(* Logix 5000 AddOnInstructionDefinition export Banner_R90C_R95C_R130C_Param_v4; software revision 33.00 *)

TYPE Banner_Hub_Discrete_Host_Out_Mirror_v4 :
STRUCT
   Mirroring_Enable : SINT;   // 0=Disabled, 1=Enabled.
   Mirroring_Port : SINT;   // 0=Port1, 1=Port2, 2=Port3, 3=Port4, Next set only for R95C 4=Port5, 5=Port6, 6=Port7, 7=Port8.
   Mirroring_Channel : SINT;   // 0=Discrete1, 1=Discrete2.
   Mirroring_Inversion : SINT;   // 0=Not Inverted, 1=Inverted.
   Mirroring_Polarity : SINT;   // 0=NPN Output, 1=PNP Output.
   Mirroring_Output_Type : SINT;   // 0=Output Open Collector, 1=Output Push Pull.
END_STRUCT
END_TYPE

TYPE Banner_Hub_IO_Metrics_v4 :
STRUCT
   Port_Discrete1_Count : DINT;
   Port_Discrete1_Duration : DINT;
   Port_Discrete1_Events_Per_Minute : DINT;
   Port_Discrete1_Totalizer : DINT;
   Port_Discrete2_Count : DINT;
   Port_Discrete2_Duration : DINT;
   Port_Discrete2_Events_Per_Minute : DINT;
   Port_Discrete2_Totalizer : DINT;
END_STRUCT
END_TYPE

TYPE Banner_Hub_Port_Config_B22_v4 :   // Data elements that are unique to the B22 version of the IO-Link Hub.
STRUCT
   Mirroring_Enable : SINT;   // 0 = Disabled, 1 = Enabled.
   Mirroring_Port_Selection : SINT;   // 0 = Port1, 1 = Port2, 2 = Port3, 3 = Prot4, 4 = Prot5, 5 = Port6, 6 = Port7, 7 = Port8.
   Mirroring_Channel_Selection : INT;   // 0 = Discrete 1, 1 = Discrete 2.
   Mirroring_Inversion : SINT;   // 0 = Not Inverted, 1 = Inverted.
END_STRUCT
END_TYPE

TYPE Banner_Hub_Port_Config_v4 :
STRUCT
   Discrete1_IO : INT;   // 0=NPN, 1=PNP
   Discrete1_Delay_Mode : INT;   // 0=Disabled,1=On Off Delay, 2=On OneShot, 3=Off OneShot, 4=On Pulse Stretcher, 5=Off Pulse Stretcher, 6=Totalizer, 7=Retriggerable On OneShot, 8=Retriggerable Off OneShot.
   Discrete1_Delay_Timer1 : DINT;
   Discrete1_Delay_Timer2 : DINT;
   Discrete1_B22_Options : Banner_Hub_Port_Config_B22_v4;
   Discrete2_IO : INT;   // 0=NPN, 1=PNP
   Discrete2_Delay_Mode : INT;   // 0=Disabled,1=On Off Delay, 2=On OneShot, 3=Off OneShot, 4=On Pulse Stretcher, 5=Off Pulse Stretcher, 6=Totalizer, 7=Retriggerable On OneShot, 8=Retriggerable Off OneShot.
   Discrete2_Delay_Timer1 : DINT;
   Discrete2_Delay_Timer2 : DINT;
   Discrete2_B22_Options : Banner_Hub_Port_Config_B22_v4;
   Mirroring_Enable : SINT;   // 0=Disabled, 1=Enabled.
   Mirroring_Port : SINT;   // 0=Port1, 1=Port2, 2=Port3, 3=Port4. Next set only for R95C 4=Port5, 5=Port6, 6=Port7, 7=Port8.
   Mirroring_Channel : SINT;   // 0=Discrete1, 1=Discrete2.
   Mirroring_Inversion : SINT;   // 0=Not Inverted, 1=Inverted.
END_STRUCT
END_TYPE

TYPE Banner_Hub_RD_v4 :   // UDT that stores the Write Data for a LM.
STRUCT
   Master_Cycle_Time : INT;
   Min_Cycle_Time : INT;
   M_Sequence_Capability : INT;
   IO_Link_Version_ID : INT;
   Process_Data_Input_Length : INT;
   Process_Data_Output_Length : INT;
   Combined_Vendor_ID : DINT;   // IO-Link Vendor ID
   Vendor_ID1 : INT;
   Vendor_ID2 : INT;
   Combined_Device_ID : DINT;   // IO-Link Device ID
   Device_ID1 : INT;
   Device_ID2 : INT;
   Device_ID3 : INT;
   Serial_Number : STRING;
   All_Time_Run_Time : DINT;   // Run Counter in 1/4 hr increments
   IO_Metrics : Banner_Hub_IO_Metrics_v4[9];
END_STRUCT
END_TYPE

TYPE Banner_Hub_SMR_Port_v4 :
STRUCT
   Discrete1 : SINT;   // 0 = Normal setting, 1 = Reset metrics.
   Discrete2 : SINT;   // 0 = Normal setting, 1 = Reset metrics.
   Discrete1_Reset_Count : DINT;   // Value that Counter is set to when a Reset Metrics operation is activated.
   Discrete2_Reset_Count : DINT;   // Value that Counter is set to when a Reset Metrics operation is activated.
END_STRUCT
END_TYPE

TYPE Banner_Hub_v4 :   // All of the parameters for a R90C, R95C, or R130C Hub.
STRUCT
   Initial_Global_Read : BOOL;   // Determines if all of the IO-Link data has been read into the PLC yet
   Command : INT;   // Value placed in here will activate a read or write to a specifc IO-Link Index
   Read : Banner_Hub_RD_v4;   // Read Only Data
   Write : Banner_Hub_WD_v4;   // Write Data
   Archive : Banner_Hub_WD_v4;   // Archive of Write Data
   Reset : BOOL;   // Resets AOI. This will force a complete parameter read of the sensor.
END_STRUCT
END_TYPE

TYPE Banner_Hub_VSC_v4 :
STRUCT
   PDin1_Metric : INT;   // 0=Disabled, 1=Count, 2=Duration, 3=Events Per Minute.
   PDin1_Port : INT;   // 0=Port 1, 1=Port 2, 2=Port 3, 3=Port 4. Only for R95 models 5=Port 6, 6=Port 7, 7=Port 8.
   PDin1_Channel : INT;   // 0=Discrete 1, 1 =Discrete 2.
   PDin2_Metric : INT;   // 0=Disabled, 1=Count, 2=Duration, 3=Events Per Minute.
   PDin2_Port : INT;   // 0=Port 1, 1=Port 2, 2=Port 3, 3=Port 4. Only for R95 models 5=Port 6, 6=Port 7, 7=Port 8.
   PDin2_Channel : INT;   // 0=Discrete 1, 1 =Discrete 2.
   PDin3_Metric : INT;   // 0=Disabled, 1=Count, 2=Duration, 3=Events Per Minute.
   PDin3_Port : INT;   // 0=Port 1, 1=Port 2, 2=Port 3, 3=Port 4. Only for R95 models 5=Port 6, 6=Port 7, 7=Port 8.
   PDin3_Channel : INT;   // 0=Discrete 1, 1 =Discrete 2.
   PDin4_Metric : INT;   // 0=Disabled, 1=Count, 2=Duration, 3=Events Per Minute.
   PDin4_Port : INT;   // 0=Port 1, 1=Port 2, 2=Port 3, 3=Port 4. Only for R95 models 5=Port 6, 6=Port 7, 7=Port 8.
   PDin4_Channel : INT;   // 0=Discrete 1, 1 =Discrete 2.
END_STRUCT
END_TYPE

TYPE Banner_Hub_WD_v4 :   // UDT that stores the Write Data for a LM.
STRUCT
   System_Command : INT;   // See IODD file for list of commands that can be activated via the System Command interface
   Parameter_Access_Lock : SINT;   // Write access to all parameters is prohibited while value is 1. Only this parameter can be adjusted when value is 1.
   Data_Storage_Lock : SINT;   // Automatic data storage is disabled when this value is equal to 1. Read access is not affected.
   Local_Parameterization_Lock : SINT;   // Parameterization via local control elements on device is disabled.
   Local_User_Interface_Lock : SINT;   // Operation of local user interface is disabled.
   Resettable_Run_Time : DINT;   // Run Counter in 1/4 hr increments
   VSC : Banner_Hub_VSC_v4;   // Vendor Specific Configuration R90C-4B21 and R95C-8B21 models.
   Process_Data_Grouping : SINT;   // R95-8B22 only. 0 = Group by Port, 1 = Group by Channel.
   All_Time_Run_Time_Event_Time : DINT;   // Event Time in 1/4 hr increments
   Resettable_Run_Time_Event_Time : DINT;   // Event Time in 1/4 hour increments
   SMR : Banner_Hub_SMR_Port_v4[10];   // Selectable Metric Reset.
   Port_Config : Banner_Hub_Port_Config_v4[10];
   Discrete_Host_Out_Mirroring : Banner_Hub_Discrete_Host_Out_Mirror_v4;
END_STRUCT
END_TYPE

TYPE Banner_IOL_Port_v4 :   // UDT that has all of the data items necessary to communicate with a specific Port on a IO-Link Master
STRUCT
   Port_Controlled : INT;   // Each bit represents a port on an IO-Link Master. Set to 1 to tell AOI to control that port.
   Port_Activate : INT;   // Each bit represents a port on an IO-Link Master. When ON that port will process any commands in queue.
   Port_Read : INT;   // Each bit represents a port on an IO-Link Master. Used to determine when device AOI has requested a Read command.
   Port_Write : INT;   // Each bit represents a port on an IO-Link Master. Used to determine when device AOI has requested a Write command.
   Port_RW_Complete : INT;   // Each bit represents a port on an IO-Link Master. Tells device AOI that Read or Write request has been completed.
   Port_Device_Read : INT;
   Data_Transfer : SINT[190];   // Array to transfer data from IO-Master to device AOIs.
END_STRUCT
END_TYPE

ADD_ON_INSTRUCTION Banner_R90C_R95C_R130C_Param_v4   (* revision 4.4, vendor Banner Engineering *)
// AOI to read and write parameter data to an IO-Link R90C-4K, R95C-8B21, R95C-8B22, or R130C-8B22 IO-Link Hub.
// Revision note:
// Added R130C.
VAR_IN_OUT
   Hub : Banner_Hub_v4; {required}
   Port_Data : Banner_IOL_Port_v4; {required}
END_VAR
VAR_INPUT
   Port : INT; {required}
   Type : INT; {required}   // 4 = R90C-4B21, 8 = R95C-8B21, 22 = R95-8B22
END_VAR
VAR
   Control : DINT; {access None}
   Global_Read_Command_Value : INT; {access None}
   Global_Write_Command_Value : INT; {access None}
   Command_Being_Processed : BOOL; {access None}
   Update_Archive : BOOL; {access None}
   Index_Write_Inprocess : INT; {access None}
   Index_Write_Control : INT; {access None}
   Temp_Excess_Gain : DINT; {access None}
   Inprocess_Index : DINT; {access None}
   Index2 : SINT; {access None}
   Index1 : SINT; {access None}
   Index4 : SINT; {access None}
   Index3 : SINT; {access None}
   Index6 : SINT; {access None}
   Index5 : SINT; {access None}
   Index7 : SINT; {access None}
END_VAR

ROUTINE Logic   (* ladder *)
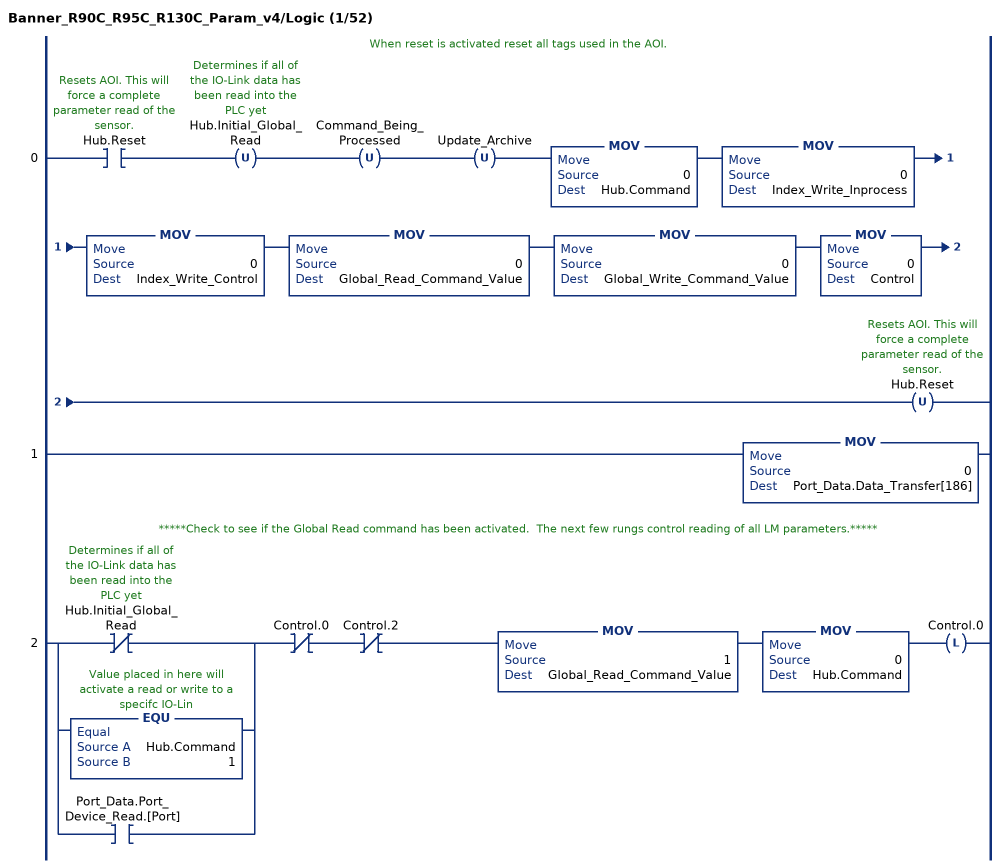
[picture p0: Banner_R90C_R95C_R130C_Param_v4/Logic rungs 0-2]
   // When reset is activated reset all tags used in the AOI.
   0: XIC(Hub.Reset)OTU(Hub.Initial_Global_Read)OTU(Command_Being_Processed)OTU(Update_Archive)MOV(0,Hub.Command)MOV(0,Index_Write_Inprocess)MOV(0,Index_Write_Control)MOV(0,Global_Read_Command_Value)MOV(0,Global_Write_Command_Value)MOV(0,Control)OTU(Hub.Reset);
   1: MOV(0,Port_Data.Data_Transfer[186]);
   // *****Check to see if the Global Read command has been activated.  The next few rungs control reading of all LM parameters.*****
   2: [XIO(Hub.Initial_Global_Read) ,EQU(Hub.Command,1) ,XIC(Port_Data.Port_Device_Read.[Port]) ]XIO(Control.0)XIO(Control.2)MOV(1,Global_Read_Command_Value)MOV(0,Hub.Command)OTL(Control.0);
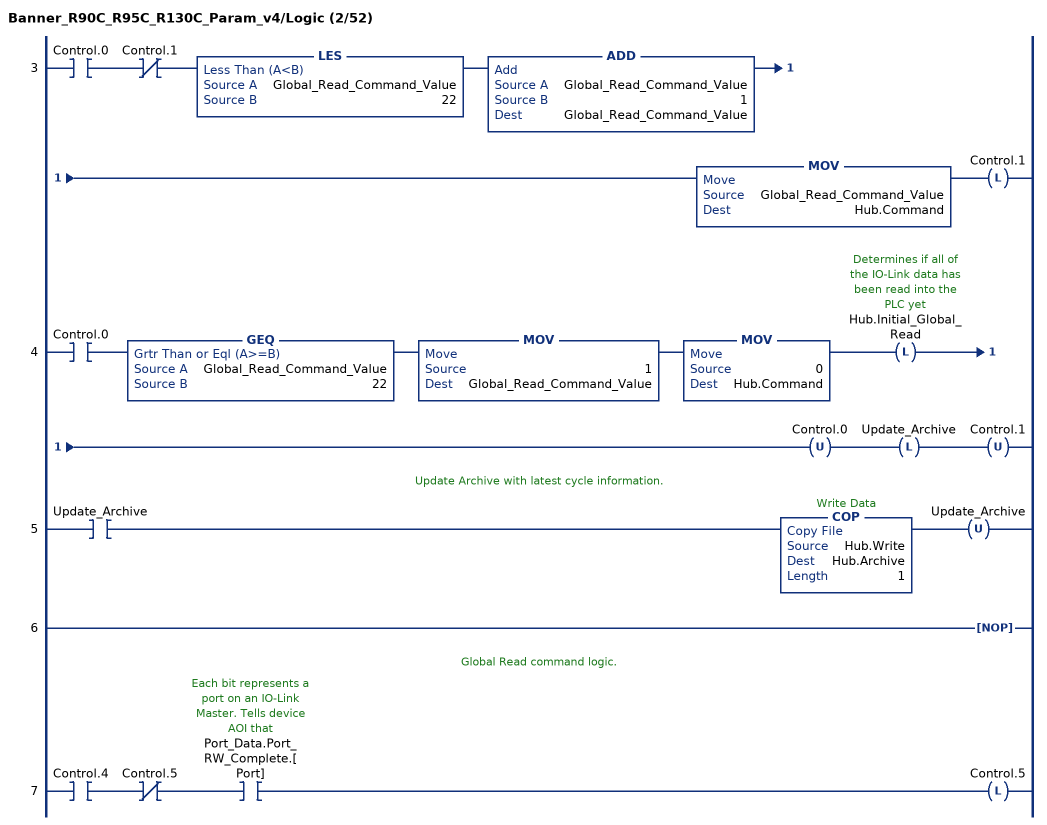
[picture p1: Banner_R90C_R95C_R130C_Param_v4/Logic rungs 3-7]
   3: XIC(Control.0)XIO(Control.1)LES(Global_Read_Command_Value,22)ADD(Global_Read_Command_Value,1,Global_Read_Command_Value)MOV(Global_Read_Command_Value,Hub.Command)OTL(Control.1);
   4: XIC(Control.0)GEQ(Global_Read_Command_Value,22)MOV(1,Global_Read_Command_Value)MOV(0,Hub.Command)OTL(Hub.Initial_Global_Read)OTU(Control.0)OTL(Update_Archive)OTU(Control.1);
   // Update Archive with latest cycle information.
   5: XIC(Update_Archive)COP(Hub.Write,Hub.Archive,1)OTU(Update_Archive);
   6: NOP();
   // Global Read command logic.
   7: XIC(Control.4)XIO(Control.5)XIC(Port_Data.Port_RW_Complete.[Port])OTL(Control.5);
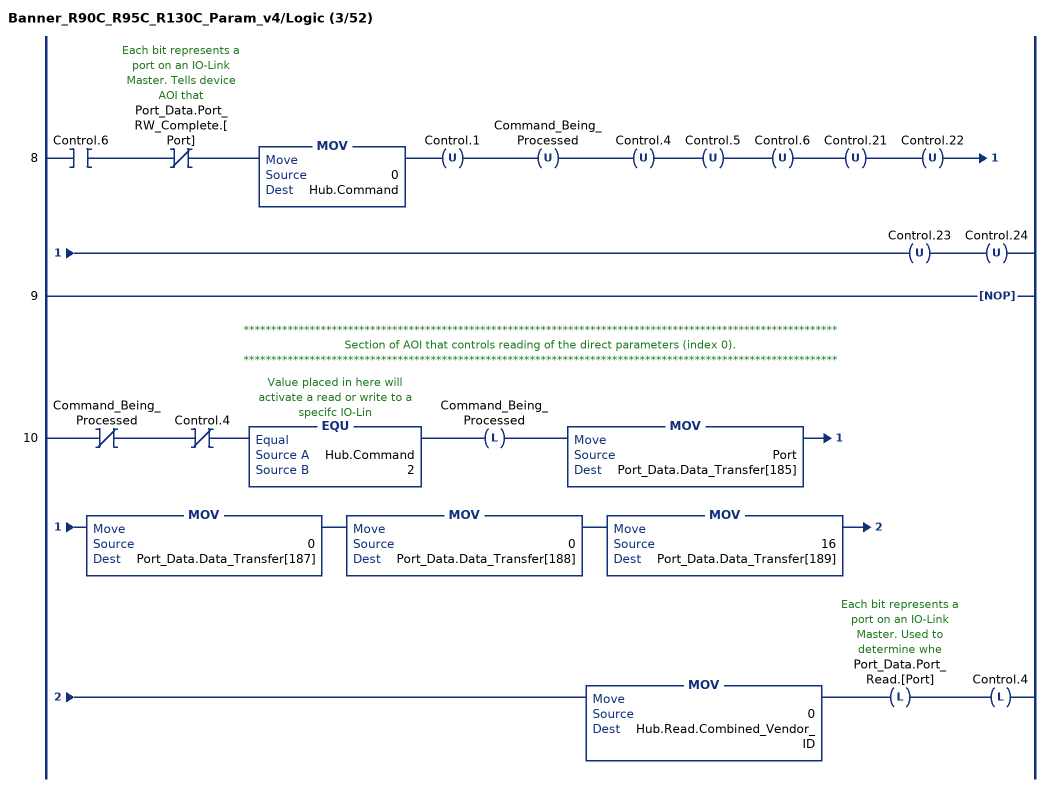
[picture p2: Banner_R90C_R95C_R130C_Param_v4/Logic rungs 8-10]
   8: XIC(Control.6)XIO(Port_Data.Port_RW_Complete.[Port])MOV(0,Hub.Command)OTU(Control.1)OTU(Command_Being_Processed)OTU(Control.4)OTU(Control.5)OTU(Control.6)OTU(Control.21)OTU(Control.22)OTU(Control.23)OTU(Control.24);
   9: NOP();
   // ************************************************************************************************************
   // Section of AOI that controls reading of the direct parameters (index 0).
   // ************************************************************************************************************
   10: XIO(Command_Being_Processed)XIO(Control.4)EQU(Hub.Command,2)OTL(Command_Being_Processed)MOV(Port,Port_Data.Data_Transfer[185])MOV(0,Port_Data.Data_Transfer[187])MOV(0,Port_Data.Data_Transfer[188])MOV(16,Port_Data.Data_Transfer[189])MOV(0,Hub.Read.Combined_Vendor_ID)OTL(Port_Data.Port_Read.[Port])OTL(Control.4);
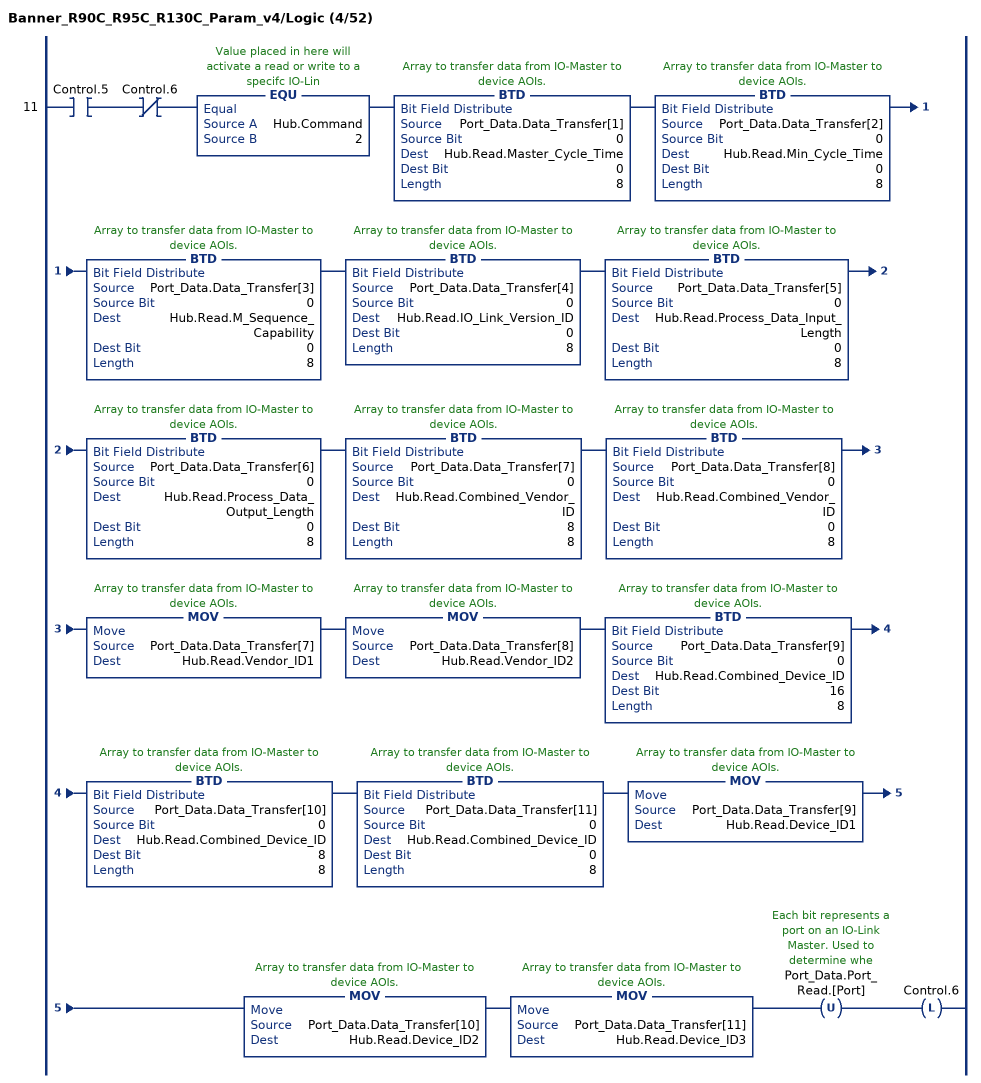
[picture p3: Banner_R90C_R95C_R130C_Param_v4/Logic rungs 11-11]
   11: XIC(Control.5)XIO(Control.6)EQU(Hub.Command,2)BTD(Port_Data.Data_Transfer[1],0,Hub.Read.Master_Cycle_Time,0,8)BTD(Port_Data.Data_Transfer[2],0,Hub.Read.Min_Cycle_Time,0,8)BTD(Port_Data.Data_Transfer[3],0,Hub.Read.M_Sequence_Capability,0,8)BTD(Port_Data.Data_Transfer[4],0,Hub.Read.IO_Link_Version_ID,0,8)BTD(Port_Data.Data_Transfer[5],0,Hub.Read.Process_Data_Input_Length,0,8)BTD(Port_Data.Data_Transfer[6],0,Hub.Read.Process_Data_Output_Length,0,8)BTD(Port_Data.Data_Transfer[7],0,Hub.Read.Combined_Vendor_ID,8,8)BTD(Port_Data.Data_Transfer[8],0,Hub.Read.Combined_Vendor_ID,0,8)MOV(Port_Data.Data_Transfer[7],Hub.Read.Vendor_ID1)MOV(Port_Data.Data_Transfer[8],Hub.Read.Vendor_ID2)BTD(Port_Data.Data_Transfer[9],0,Hub.Read.Combined_Device_ID,16,8)BTD(Port_Data.Data_Transfer[10],0,Hub.Read.Combined_Device_ID,8,8)BTD(Port_Data.Data_Transfer[11],0,Hub.Read.Combined_Device_ID,0,8)MOV(Port_Data.Data_Transfer[9],Hub.Read.Device_ID1)MOV(Port_Data.Data_Transfer[10],Hub.Read.Device_ID2)MOV(Port_Data.Data_Transfer[11],Hub.Read.Device_ID3)OTU(Port_Data.Port_Read.[Port])OTL(Control.6);
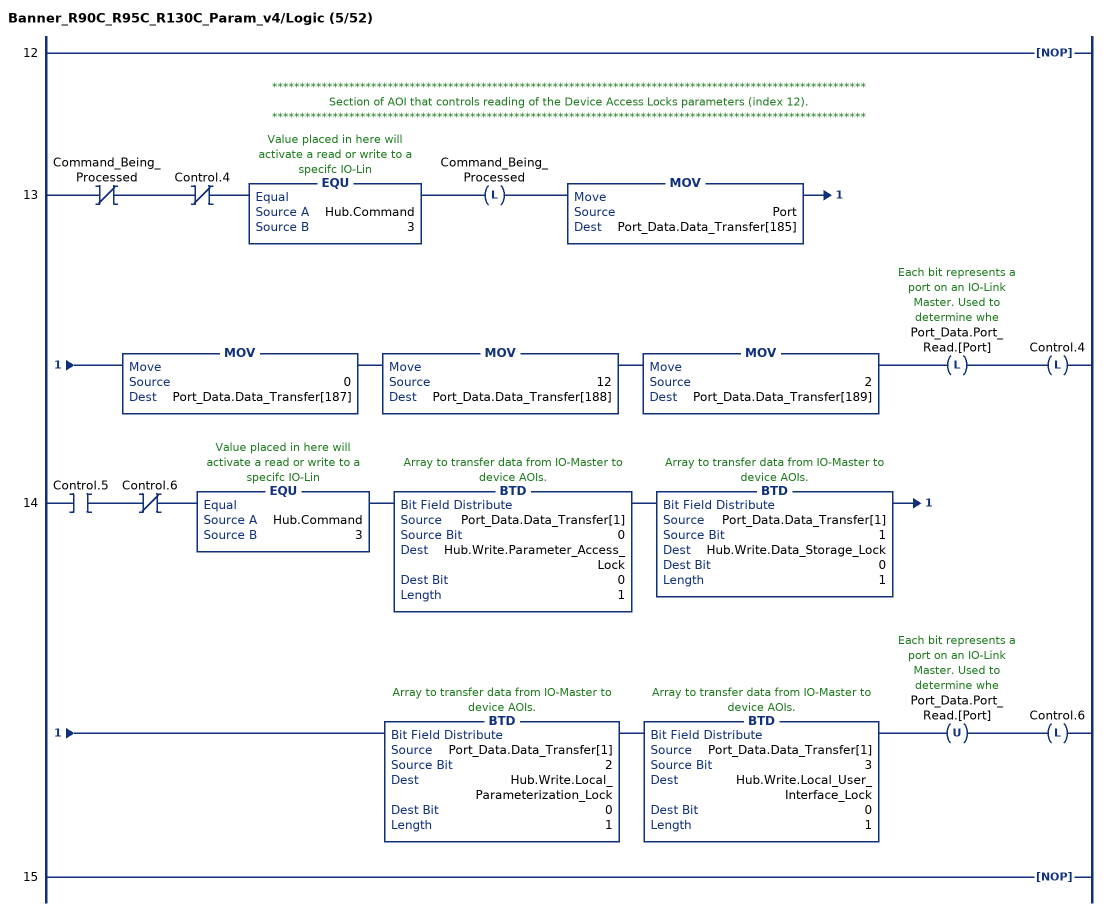
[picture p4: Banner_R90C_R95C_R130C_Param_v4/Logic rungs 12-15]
   12: NOP();
   // ************************************************************************************************************
   // Section of AOI that controls reading of the Device Access Locks parameters (index 12).
   // ************************************************************************************************************
   13: XIO(Command_Being_Processed)XIO(Control.4)EQU(Hub.Command,3)OTL(Command_Being_Processed)MOV(Port,Port_Data.Data_Transfer[185])MOV(0,Port_Data.Data_Transfer[187])MOV(12,Port_Data.Data_Transfer[188])MOV(2,Port_Data.Data_Transfer[189])OTL(Port_Data.Port_Read.[Port])OTL(Control.4);
   14: XIC(Control.5)XIO(Control.6)EQU(Hub.Command,3)BTD(Port_Data.Data_Transfer[1],0,Hub.Write.Parameter_Access_Lock,0,1)BTD(Port_Data.Data_Transfer[1],1,Hub.Write.Data_Storage_Lock,0,1)BTD(Port_Data.Data_Transfer[1],2,Hub.Write.Local_Parameterization_Lock,0,1)BTD(Port_Data.Data_Transfer[1],3,Hub.Write.Local_User_Interface_Lock,0,1)OTU(Port_Data.Port_Read.[Port])OTL(Control.6);
   15: NOP();
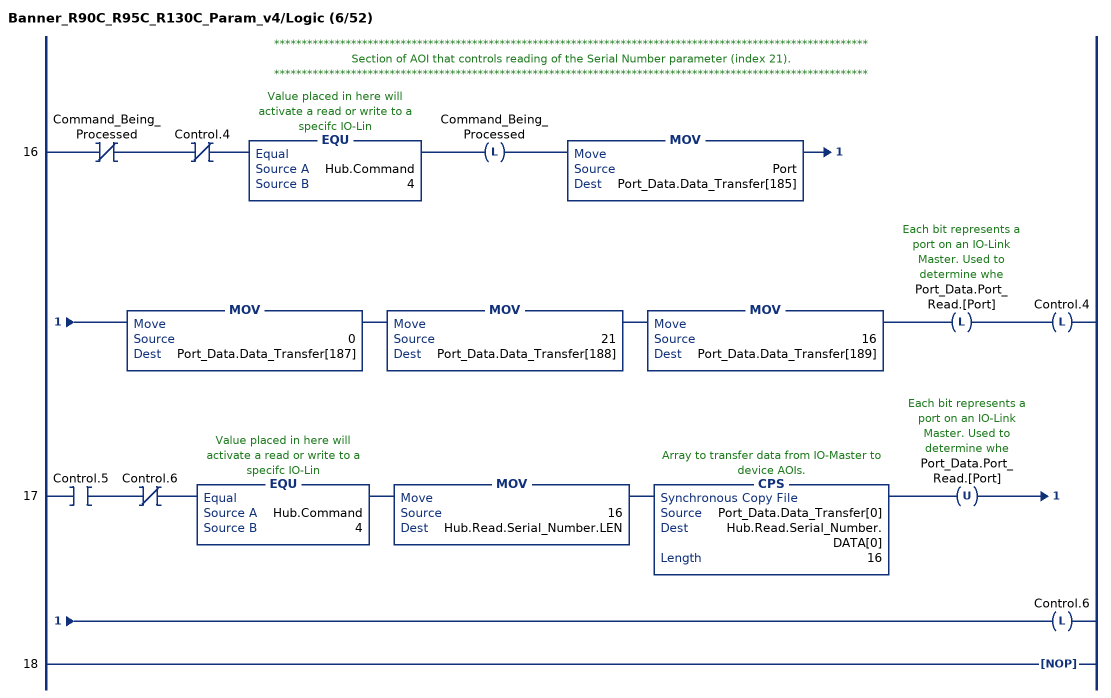
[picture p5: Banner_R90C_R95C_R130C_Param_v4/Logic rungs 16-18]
   // ************************************************************************************************************
   // Section of AOI that controls reading of the Serial Number parameter (index 21).
   // ************************************************************************************************************
   16: XIO(Command_Being_Processed)XIO(Control.4)EQU(Hub.Command,4)OTL(Command_Being_Processed)MOV(Port,Port_Data.Data_Transfer[185])MOV(0,Port_Data.Data_Transfer[187])MOV(21,Port_Data.Data_Transfer[188])MOV(16,Port_Data.Data_Transfer[189])OTL(Port_Data.Port_Read.[Port])OTL(Control.4);
   17: XIC(Control.5)XIO(Control.6)EQU(Hub.Command,4)MOV(16,Hub.Read.Serial_Number.LEN)CPS(Port_Data.Data_Transfer[0],Hub.Read.Serial_Number.DATA[0],16)OTU(Port_Data.Port_Read.[Port])OTL(Control.6);
   18: NOP();
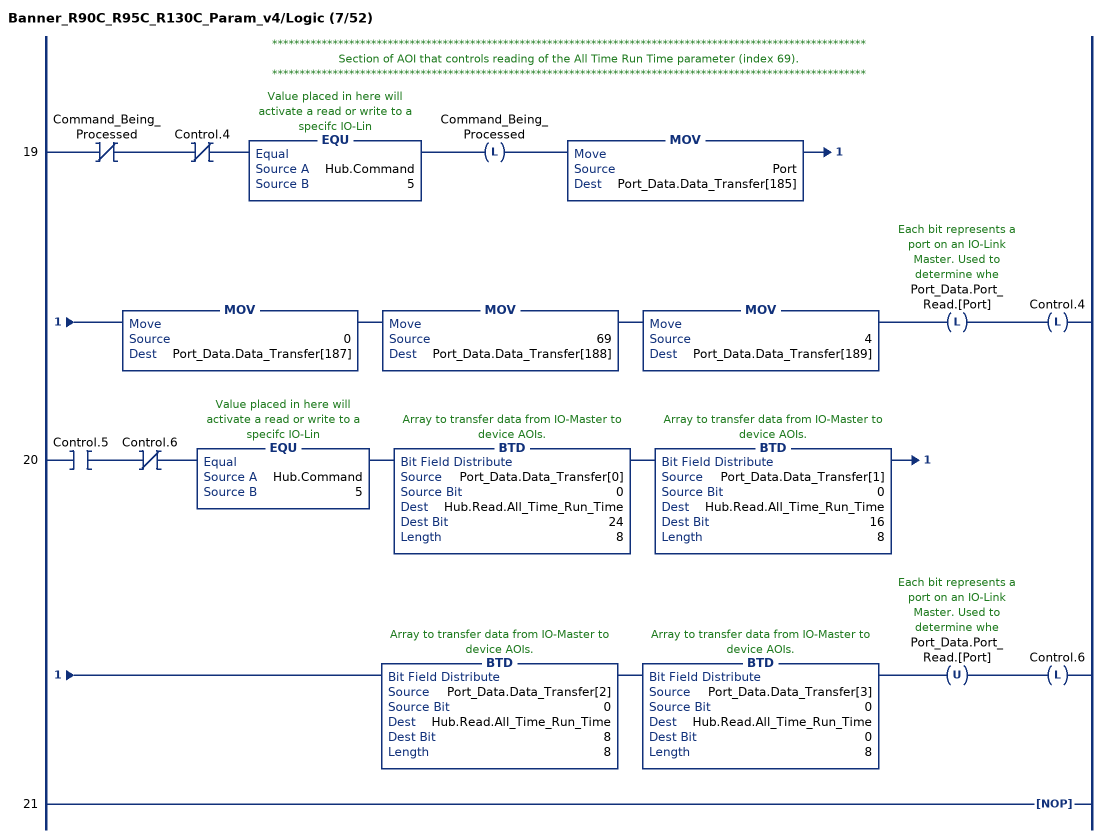
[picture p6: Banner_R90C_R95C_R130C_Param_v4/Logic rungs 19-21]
   // ************************************************************************************************************
   // Section of AOI that controls reading of the All Time Run Time parameter (index 69).
   // ************************************************************************************************************
   19: XIO(Command_Being_Processed)XIO(Control.4)EQU(Hub.Command,5)OTL(Command_Being_Processed)MOV(Port,Port_Data.Data_Transfer[185])MOV(0,Port_Data.Data_Transfer[187])MOV(69,Port_Data.Data_Transfer[188])MOV(4,Port_Data.Data_Transfer[189])OTL(Port_Data.Port_Read.[Port])OTL(Control.4);
   20: XIC(Control.5)XIO(Control.6)EQU(Hub.Command,5)BTD(Port_Data.Data_Transfer[0],0,Hub.Read.All_Time_Run_Time,24,8)BTD(Port_Data.Data_Transfer[1],0,Hub.Read.All_Time_Run_Time,16,8)BTD(Port_Data.Data_Transfer[2],0,Hub.Read.All_Time_Run_Time,8,8)BTD(Port_Data.Data_Transfer[3],0,Hub.Read.All_Time_Run_Time,0,8)OTU(Port_Data.Port_Read.[Port])OTL(Control.6);
   21: NOP();
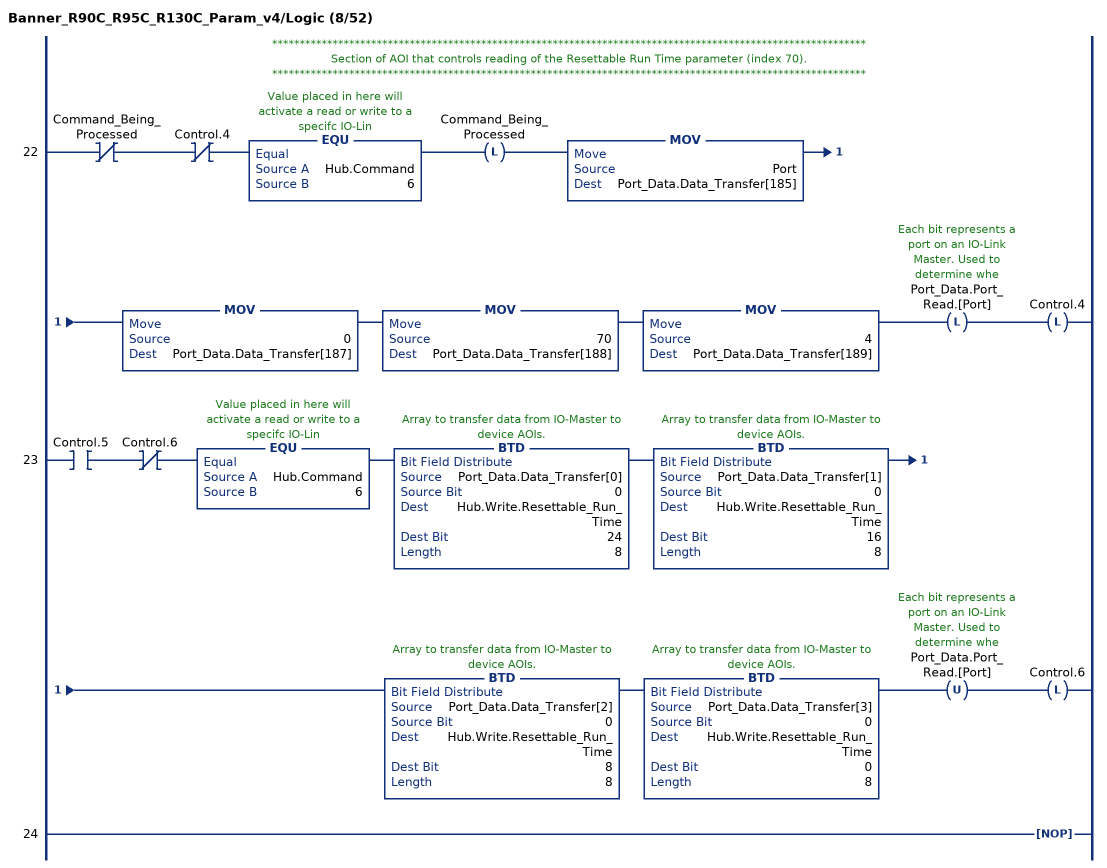
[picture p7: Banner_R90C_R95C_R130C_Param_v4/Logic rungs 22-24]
   // ************************************************************************************************************
   // Section of AOI that controls reading of the Resettable Run Time parameter (index 70).
   // ************************************************************************************************************
   22: XIO(Command_Being_Processed)XIO(Control.4)EQU(Hub.Command,6)OTL(Command_Being_Processed)MOV(Port,Port_Data.Data_Transfer[185])MOV(0,Port_Data.Data_Transfer[187])MOV(70,Port_Data.Data_Transfer[188])MOV(4,Port_Data.Data_Transfer[189])OTL(Port_Data.Port_Read.[Port])OTL(Control.4);
   23: XIC(Control.5)XIO(Control.6)EQU(Hub.Command,6)BTD(Port_Data.Data_Transfer[0],0,Hub.Write.Resettable_Run_Time,24,8)BTD(Port_Data.Data_Transfer[1],0,Hub.Write.Resettable_Run_Time,16,8)BTD(Port_Data.Data_Transfer[2],0,Hub.Write.Resettable_Run_Time,8,8)BTD(Port_Data.Data_Transfer[3],0,Hub.Write.Resettable_Run_Time,0,8)OTU(Port_Data.Port_Read.[Port])OTL(Control.6);
   24: NOP();
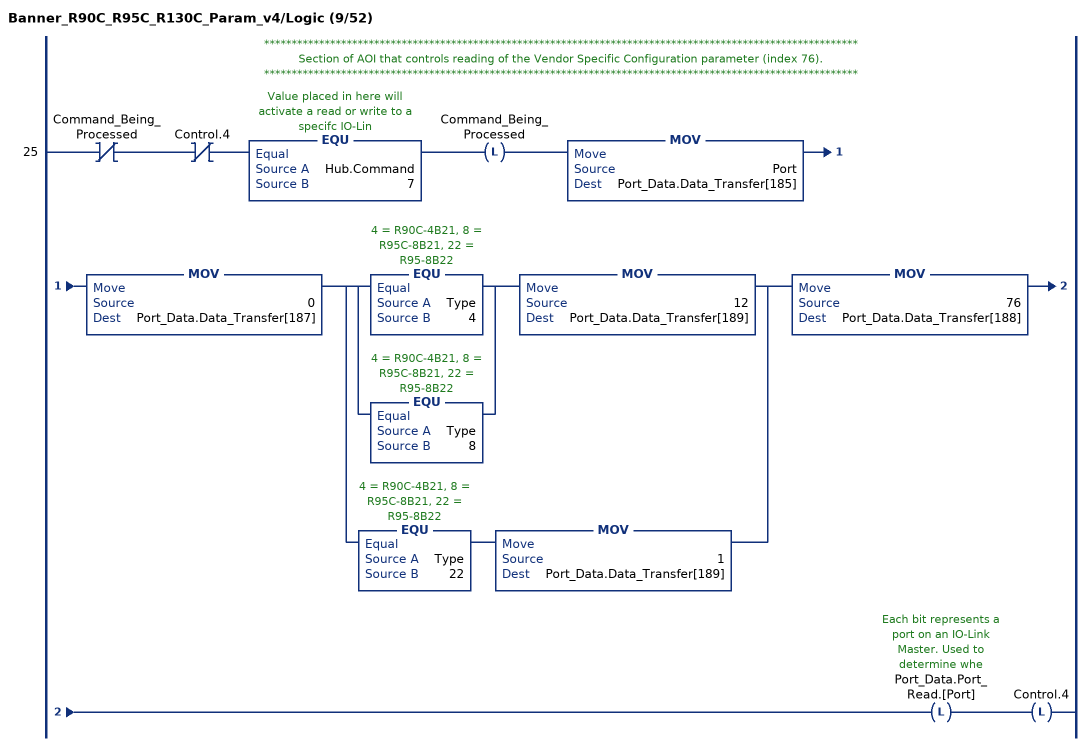
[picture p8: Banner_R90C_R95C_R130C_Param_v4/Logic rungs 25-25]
   // ************************************************************************************************************
   // Section of AOI that controls reading of the Vendor Specific Configuration parameter (index 76).
   // ************************************************************************************************************
   25: XIO(Command_Being_Processed)XIO(Control.4)EQU(Hub.Command,7)OTL(Command_Being_Processed)MOV(Port,Port_Data.Data_Transfer[185])MOV(0,Port_Data.Data_Transfer[187])[[EQU(Type,4) ,EQU(Type,8) ] MOV(12,Port_Data.Data_Transfer[189]) ,EQU(Type,22) MOV(1,Port_Data.Data_Transfer[189]) ]MOV(76,Port_Data.Data_Transfer[188])OTL(Port_Data.Port_Read.[Port])OTL(Control.4);
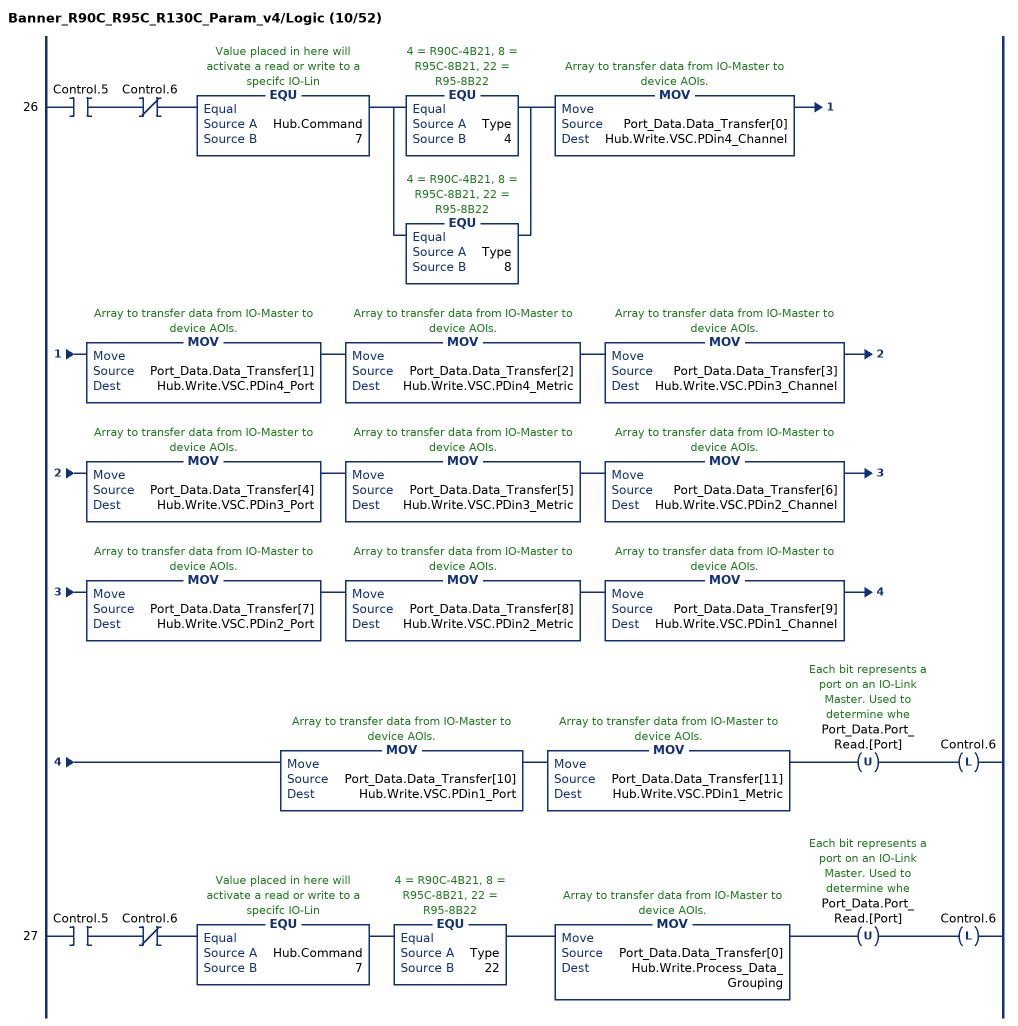
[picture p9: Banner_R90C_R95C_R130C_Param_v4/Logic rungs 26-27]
   26: XIC(Control.5)XIO(Control.6)EQU(Hub.Command,7)[EQU(Type,4) ,EQU(Type,8) ]MOV(Port_Data.Data_Transfer[0],Hub.Write.VSC.PDin4_Channel)MOV(Port_Data.Data_Transfer[1],Hub.Write.VSC.PDin4_Port)MOV(Port_Data.Data_Transfer[2],Hub.Write.VSC.PDin4_Metric)MOV(Port_Data.Data_Transfer[3],Hub.Write.VSC.PDin3_Channel)MOV(Port_Data.Data_Transfer[4],Hub.Write.VSC.PDin3_Port)MOV(Port_Data.Data_Transfer[5],Hub.Write.VSC.PDin3_Metric)MOV(Port_Data.Data_Transfer[6],Hub.Write.VSC.PDin2_Channel)MOV(Port_Data.Data_Transfer[7],Hub.Write.VSC.PDin2_Port)MOV(Port_Data.Data_Transfer[8],Hub.Write.VSC.PDin2_Metric)MOV(Port_Data.Data_Transfer[9],Hub.Write.VSC.PDin1_Channel)MOV(Port_Data.Data_Transfer[10],Hub.Write.VSC.PDin1_Port)MOV(Port_Data.Data_Transfer[11],Hub.Write.VSC.PDin1_Metric)OTU(Port_Data.Port_Read.[Port])OTL(Control.6);
   27: XIC(Control.5)XIO(Control.6)EQU(Hub.Command,7)EQU(Type,22)MOV(Port_Data.Data_Transfer[0],Hub.Write.Process_Data_Grouping)OTU(Port_Data.Port_Read.[Port])OTL(Control.6);
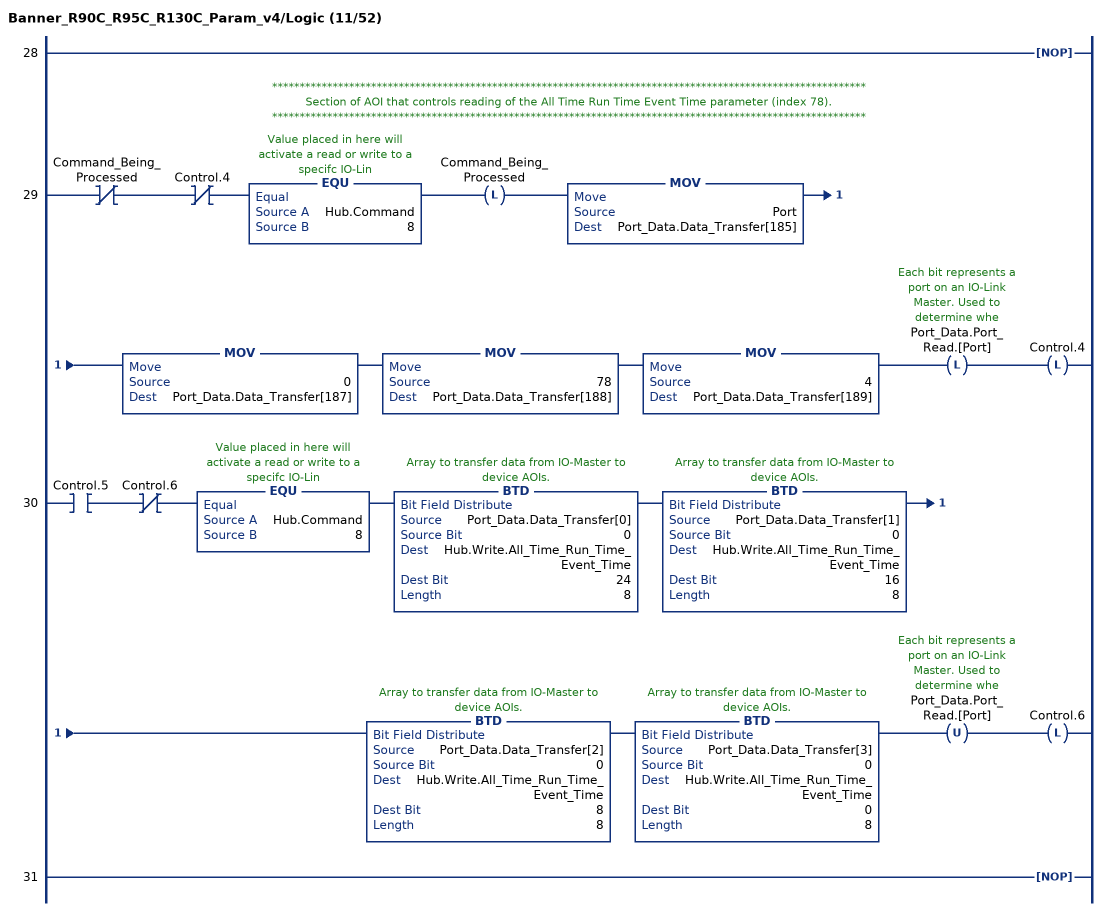
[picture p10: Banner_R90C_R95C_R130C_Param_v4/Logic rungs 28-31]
   28: NOP();
   // ************************************************************************************************************
   // Section of AOI that controls reading of the All Time Run Time Event Time parameter (index 78).
   // ************************************************************************************************************
   29: XIO(Command_Being_Processed)XIO(Control.4)EQU(Hub.Command,8)OTL(Command_Being_Processed)MOV(Port,Port_Data.Data_Transfer[185])MOV(0,Port_Data.Data_Transfer[187])MOV(78,Port_Data.Data_Transfer[188])MOV(4,Port_Data.Data_Transfer[189])OTL(Port_Data.Port_Read.[Port])OTL(Control.4);
   30: XIC(Control.5)XIO(Control.6)EQU(Hub.Command,8)BTD(Port_Data.Data_Transfer[0],0,Hub.Write.All_Time_Run_Time_Event_Time,24,8)BTD(Port_Data.Data_Transfer[1],0,Hub.Write.All_Time_Run_Time_Event_Time,16,8)BTD(Port_Data.Data_Transfer[2],0,Hub.Write.All_Time_Run_Time_Event_Time,8,8)BTD(Port_Data.Data_Transfer[3],0,Hub.Write.All_Time_Run_Time_Event_Time,0,8)OTU(Port_Data.Port_Read.[Port])OTL(Control.6);
   31: NOP();
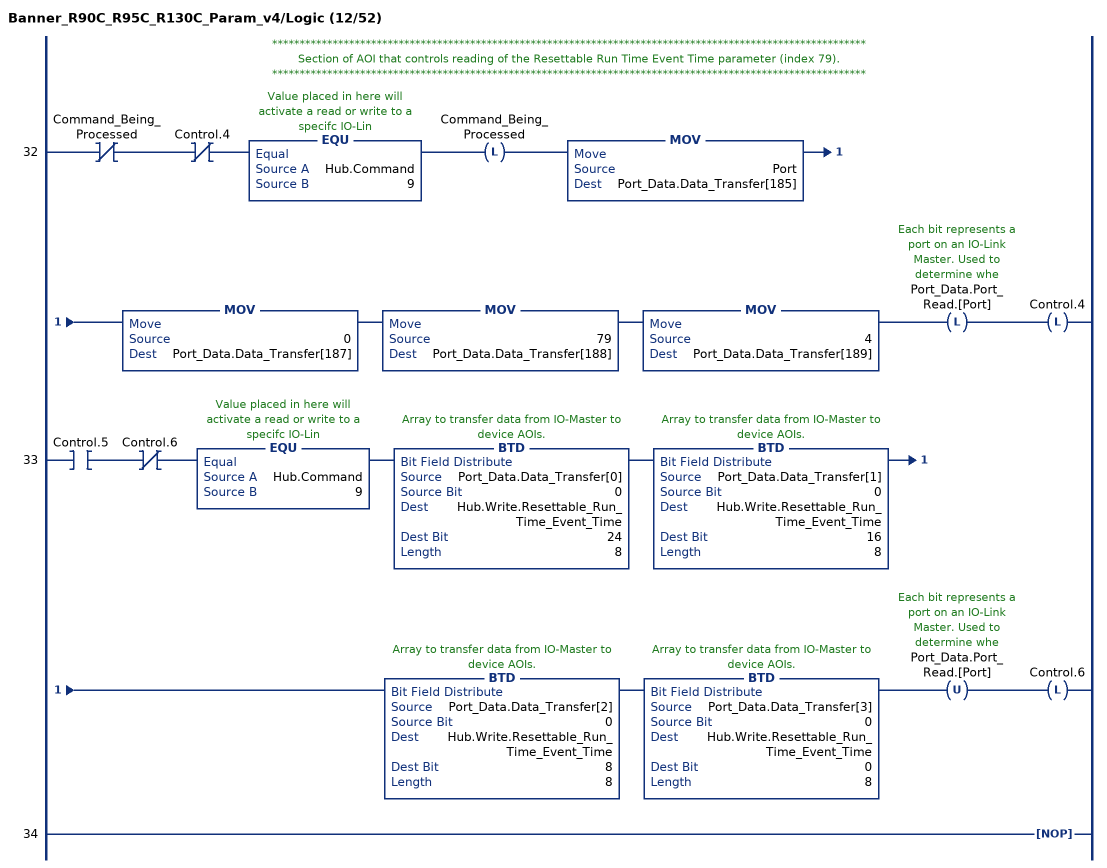
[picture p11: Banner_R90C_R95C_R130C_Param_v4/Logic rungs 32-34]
   // ************************************************************************************************************
   // Section of AOI that controls reading of the Resettable Run Time Event Time parameter (index 79).
   // ************************************************************************************************************
   32: XIO(Command_Being_Processed)XIO(Control.4)EQU(Hub.Command,9)OTL(Command_Being_Processed)MOV(Port,Port_Data.Data_Transfer[185])MOV(0,Port_Data.Data_Transfer[187])MOV(79,Port_Data.Data_Transfer[188])MOV(4,Port_Data.Data_Transfer[189])OTL(Port_Data.Port_Read.[Port])OTL(Control.4);
   33: XIC(Control.5)XIO(Control.6)EQU(Hub.Command,9)BTD(Port_Data.Data_Transfer[0],0,Hub.Write.Resettable_Run_Time_Event_Time,24,8)BTD(Port_Data.Data_Transfer[1],0,Hub.Write.Resettable_Run_Time_Event_Time,16,8)BTD(Port_Data.Data_Transfer[2],0,Hub.Write.Resettable_Run_Time_Event_Time,8,8)BTD(Port_Data.Data_Transfer[3],0,Hub.Write.Resettable_Run_Time_Event_Time,0,8)OTU(Port_Data.Port_Read.[Port])OTL(Control.6);
   34: NOP();
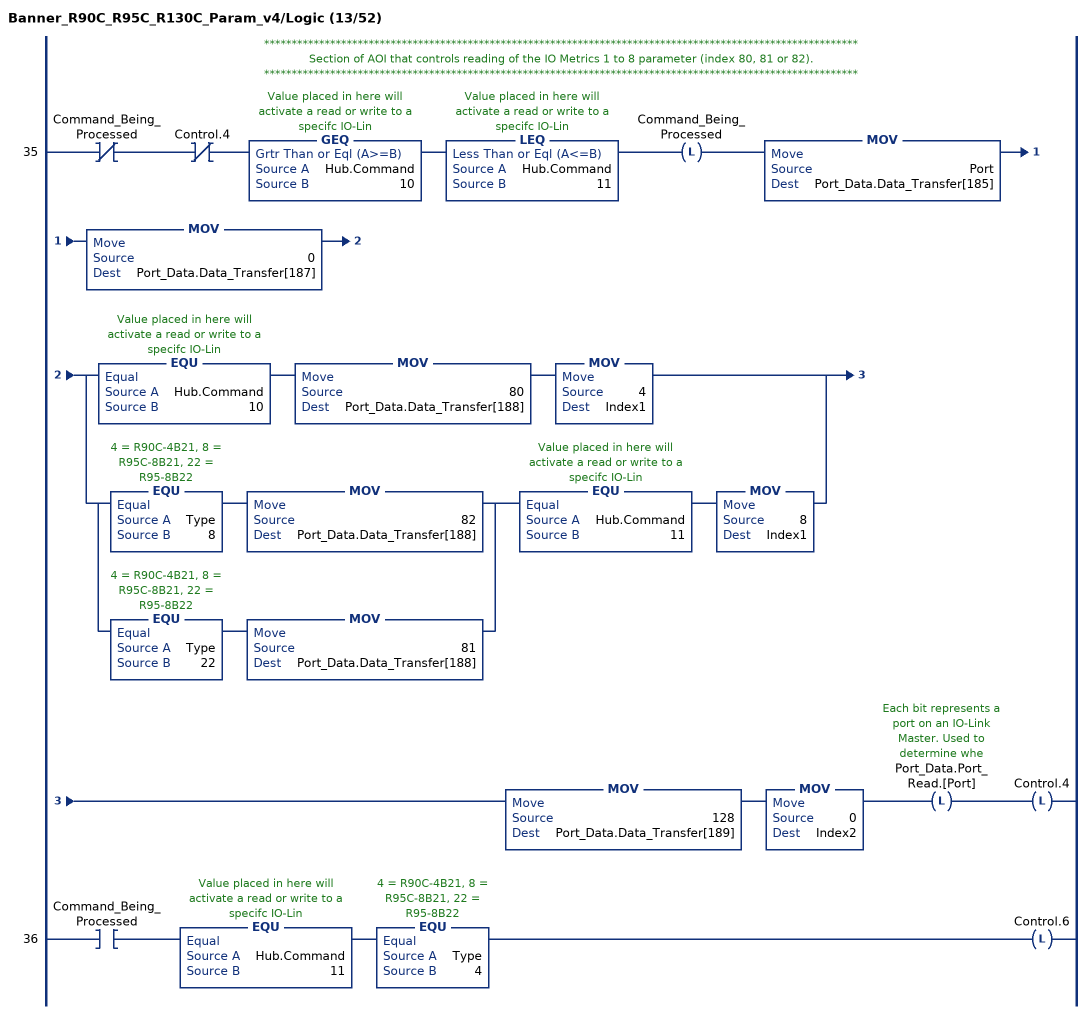
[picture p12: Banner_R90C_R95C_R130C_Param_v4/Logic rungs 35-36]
   // ************************************************************************************************************
   // Section of AOI that controls reading of the IO Metrics 1 to 8 parameter (index 80, 81 or 82).
   // ************************************************************************************************************
   35: XIO(Command_Being_Processed)XIO(Control.4)GEQ(Hub.Command,10)LEQ(Hub.Command,11)OTL(Command_Being_Processed)MOV(Port,Port_Data.Data_Transfer[185])MOV(0,Port_Data.Data_Transfer[187])[EQU(Hub.Command,10) MOV(80,Port_Data.Data_Transfer[188]) MOV(4,Index1) ,[EQU(Type,8) MOV(82,Port_Data.Data_Transfer[188]) ,EQU(Type,22) MOV(81,Port_Data.Data_Transfer[188]) ] EQU(Hub.Command,11) MOV(8,Index1) ]MOV(128,Port_Data.Data_Transfer[189])MOV(0,Index2)OTL(Port_Data.Port_Read.[Port])OTL(Control.4);
   36: XIC(Command_Being_Processed)EQU(Hub.Command,11)EQU(Type,4)OTL(Control.6);
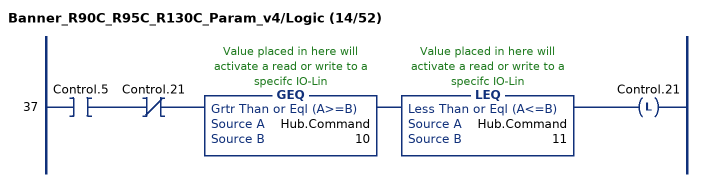
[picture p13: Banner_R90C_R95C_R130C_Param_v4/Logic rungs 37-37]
   37: XIC(Control.5)XIO(Control.21)GEQ(Hub.Command,10)LEQ(Hub.Command,11)OTL(Control.21);
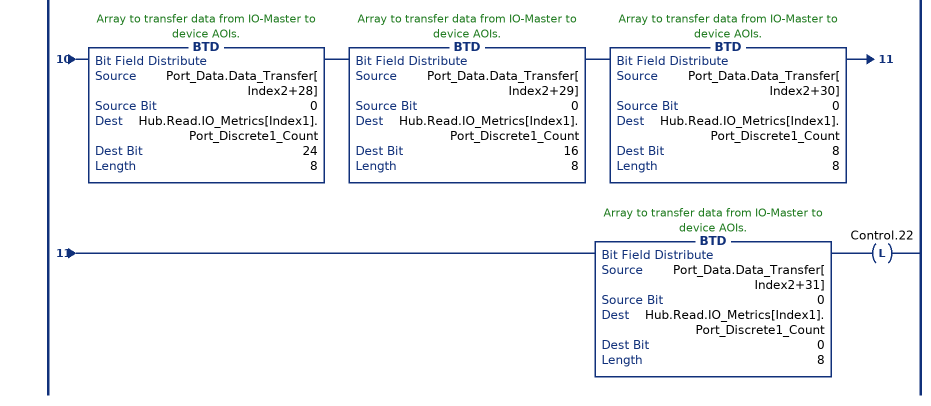
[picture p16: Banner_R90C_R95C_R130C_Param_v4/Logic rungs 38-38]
   38: XIC(Control.21)XIO(Control.22)GEQ(Hub.Command,10)LEQ(Hub.Command,11)BTD(Port_Data.Data_Transfer[Index2],0,Hub.Read.IO_Metrics[Index1].Port_Discrete2_Totalizer,24,8)BTD(Port_Data.Data_Transfer[Index2+1],0,Hub.Read.IO_Metrics[Index1].Port_Discrete2_Totalizer,16,8)BTD(Port_Data.Data_Transfer[Index2+2],0,Hub.Read.IO_Metrics[Index1].Port_Discrete2_Totalizer,8,8)BTD(Port_Data.Data_Transfer[Index2+3],0,Hub.Read.IO_Metrics[Index1].Port_Discrete2_Totalizer,0,8)BTD(Port_Data.Data_Transfer[Index2+4],0,Hub.Read.IO_Metrics[Index1].Port_Discrete2_Events_Per_Minute,24,8)BTD(Port_Data.Data_Transfer[Index2+5],0,Hub.Read.IO_Metrics[Index1].Port_Discrete2_Events_Per_Minute,16,8)BTD(Port_Data.Data_Transfer[Index2+6],0,Hub.Read.IO_Metrics[Index1].Port_Discrete2_Events_Per_Minute,8,8)BTD(Port_Data.Data_Transfer[Index2+7],0,Hub.Read.IO_Metrics[Index1].Port_Discrete2_Events_Per_Minute,0,8)BTD(Port_Data.Data_Transfer[Index2+8],0,Hub.Read.IO_Metrics[Index1].Port_Discrete2_Duration,24,8)BTD(Port_Data.Data_Transfer[Index2+9],0,Hub.Read.IO_Metrics[Index1].Port_Discrete2_Duration,16,8)BTD(Port_Data.Data_Transfer[Index2+10],0,Hub.Read.IO_Metrics[Index1].Port_Discrete2_Duration,8,8)BTD(Port_Data.Data_Transfer[Index2+11],0,Hub.Read.IO_Metrics[Index1].Port_Discrete2_Duration,0,8)BTD(Port_Data.Data_Transfer[Index2+12],0,Hub.Read.IO_Metrics[Index1].Port_Discrete2_Count,24,8)BTD(Port_Data.Data_Transfer[Index2+13],0,Hub.Read.IO_Metrics[Index1].Port_Discrete2_Count,16,8)BTD(Port_Data.Data_Transfer[Index2+14],0,Hub.Read.IO_Metrics[Index1].Port_Discrete2_Count,8,8)BTD(Port_Data.Data_Transfer[Index2+15],0,Hub.Read.IO_Metrics[Index1].Port_Discrete2_Count,0,8)BTD(Port_Data.Data_Transfer[Index2+16],0,Hub.Read.IO_Metrics[Index1].Port_Discrete1_Totalizer,24,8)BTD(Port_Data.Data_Transfer[Index2+17],0,Hub.Read.IO_Metrics[Index1].Port_Discrete1_Totalizer,16,8)BTD(Port_Data.Data_Transfer[Index2+18],0,Hub.Read.IO_Metrics[Index1].Port_Discrete1_Totalizer,8,8)BTD(Port_Data.Data_Transfer[Index2+19],0,Hub.Read.IO_Metrics[Index1].Port_Discrete1_Totalizer,0,8)BTD(Port_Data.Data_Transfer[Index2+20],0,Hub.Read.IO_Metrics[Index1].Port_Discrete1_Events_Per_Minute,24,8)BTD(Port_Data.Data_Transfer[Index2+21],0,Hub.Read.IO_Metrics[Index1].Port_Discrete1_Events_Per_Minute,16,8)BTD(Port_Data.Data_Transfer[Index2+22],0,Hub.Read.IO_Metrics[Index1].Port_Discrete1_Events_Per_Minute,8,8)BTD(Port_Data.Data_Transfer[Index2+23],0,Hub.Read.IO_Metrics[Index1].Port_Discrete1_Events_Per_Minute,0,8)BTD(Port_Data.Data_Transfer[Index2+24],0,Hub.Read.IO_Metrics[Index1].Port_Discrete1_Duration,24,8)BTD(Port_Data.Data_Transfer[Index2+25],0,Hub.Read.IO_Metrics[Index1].Port_Discrete1_Duration,16,8)BTD(Port_Data.Data_Transfer[Index2+26],0,Hub.Read.IO_Metrics[Index1].Port_Discrete1_Duration,8,8)BTD(Port_Data.Data_Transfer[Index2+27],0,Hub.Read.IO_Metrics[Index1].Port_Discrete1_Duration,0,8)BTD(Port_Data.Data_Transfer[Index2+28],0,Hub.Read.IO_Metrics[Index1].Port_Discrete1_Count,24,8)BTD(Port_Data.Data_Transfer[Index2+29],0,Hub.Read.IO_Metrics[Index1].Port_Discrete1_Count,16,8)BTD(Port_Data.Data_Transfer[Index2+30],0,Hub.Read.IO_Metrics[Index1].Port_Discrete1_Count,8,8)BTD(Port_Data.Data_Transfer[Index2+31],0,Hub.Read.IO_Metrics[Index1].Port_Discrete1_Count,0,8)OTL(Control.22);
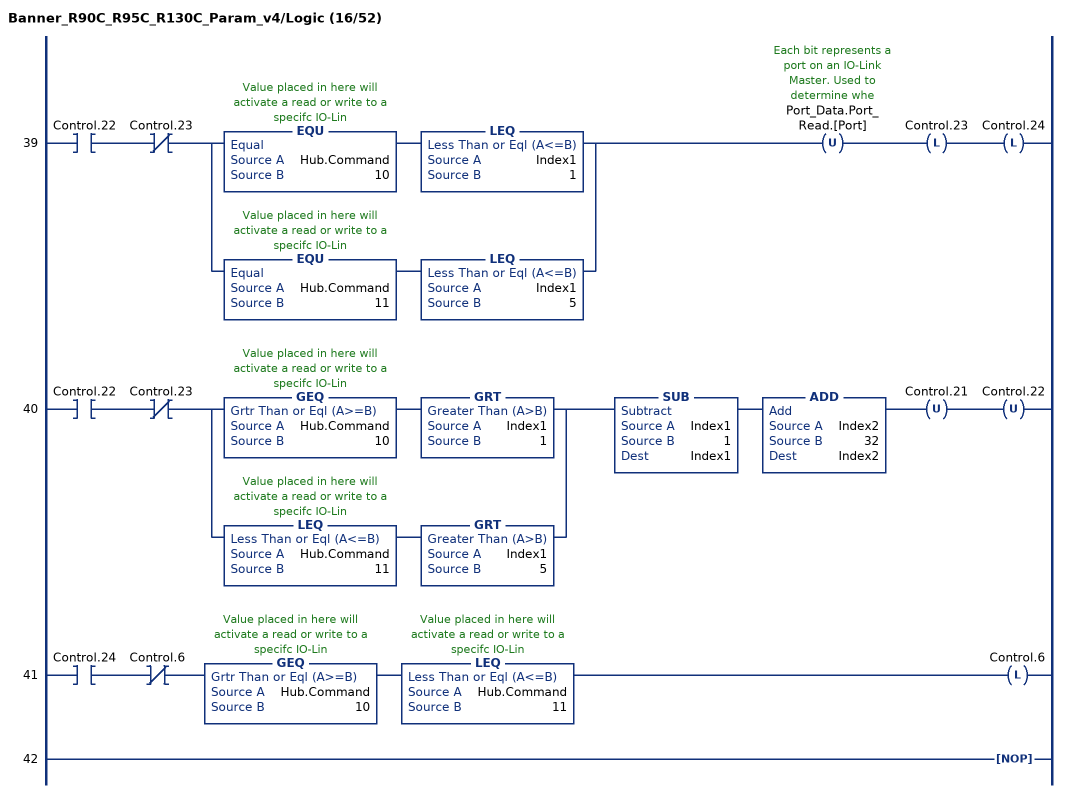
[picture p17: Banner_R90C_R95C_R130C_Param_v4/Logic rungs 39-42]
   39: XIC(Control.22)XIO(Control.23)[EQU(Hub.Command,10) LEQ(Index1,1) ,EQU(Hub.Command,11) LEQ(Index1,5) ]OTU(Port_Data.Port_Read.[Port])OTL(Control.23)OTL(Control.24);
   40: XIC(Control.22)XIO(Control.23)[GEQ(Hub.Command,10) GRT(Index1,1) ,LEQ(Hub.Command,11) GRT(Index1,5) ]SUB(Index1,1,Index1)ADD(Index2,32,Index2)OTU(Control.21)OTU(Control.22);
   41: XIC(Control.24)XIO(Control.6)GEQ(Hub.Command,10)LEQ(Hub.Command,11)OTL(Control.6);
   42: NOP();
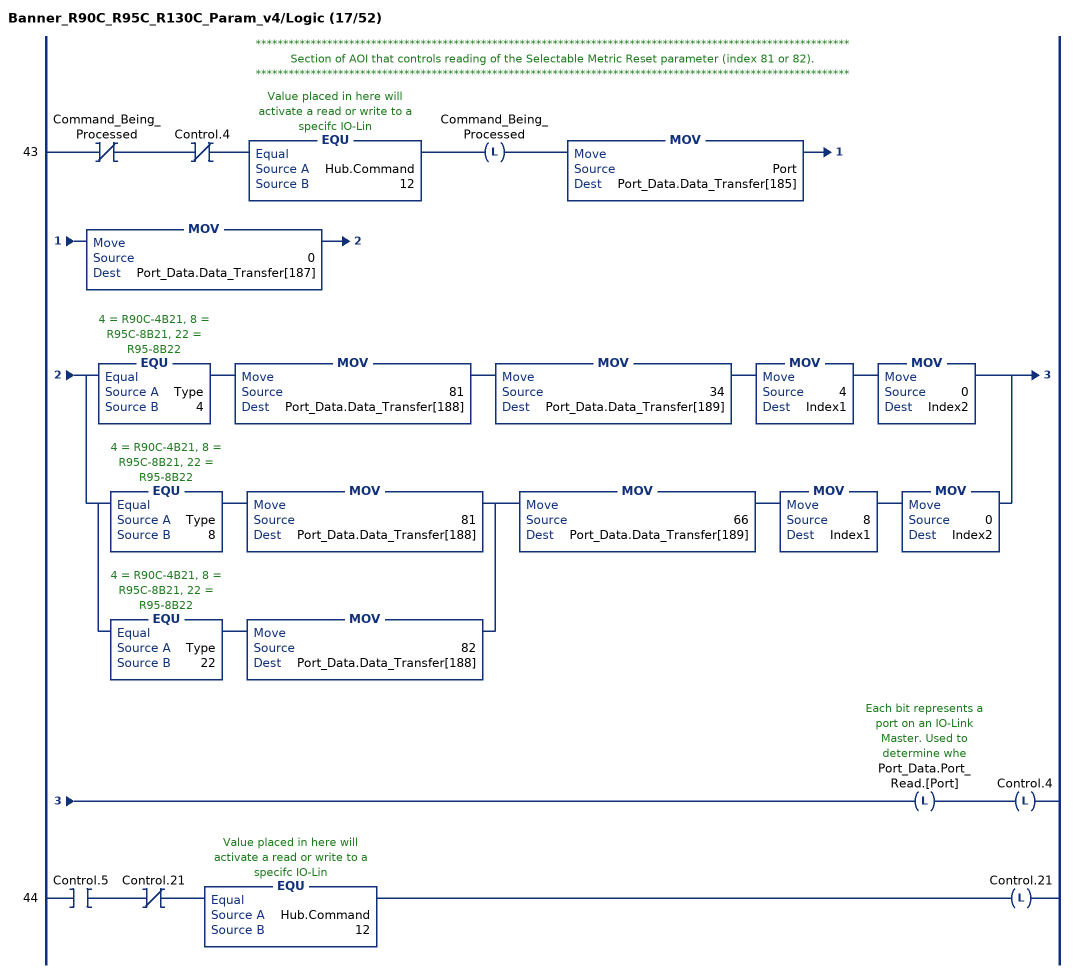
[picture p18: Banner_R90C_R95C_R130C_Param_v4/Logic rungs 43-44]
   // ************************************************************************************************************
   // Section of AOI that controls reading of the Selectable Metric Reset parameter (index 81 or 82).
   // ************************************************************************************************************
   43: XIO(Command_Being_Processed)XIO(Control.4)EQU(Hub.Command,12)OTL(Command_Being_Processed)MOV(Port,Port_Data.Data_Transfer[185])MOV(0,Port_Data.Data_Transfer[187])[EQU(Type,4) MOV(81,Port_Data.Data_Transfer[188]) MOV(34,Port_Data.Data_Transfer[189]) MOV(4,Index1) MOV(0,Index2) ,[EQU(Type,8) MOV(81,Port_Data.Data_Transfer[188]) ,EQU(Type,22) MOV(82,Port_Data.Data_Transfer[188]) ] MOV(66,Port_Data.Data_Transfer[189]) MOV(8,Index1) MOV(0,Index2) ]OTL(Port_Data.Port_Read.[Port])OTL(Control.4);
   44: XIC(Control.5)XIO(Control.21)EQU(Hub.Command,12)OTL(Control.21);
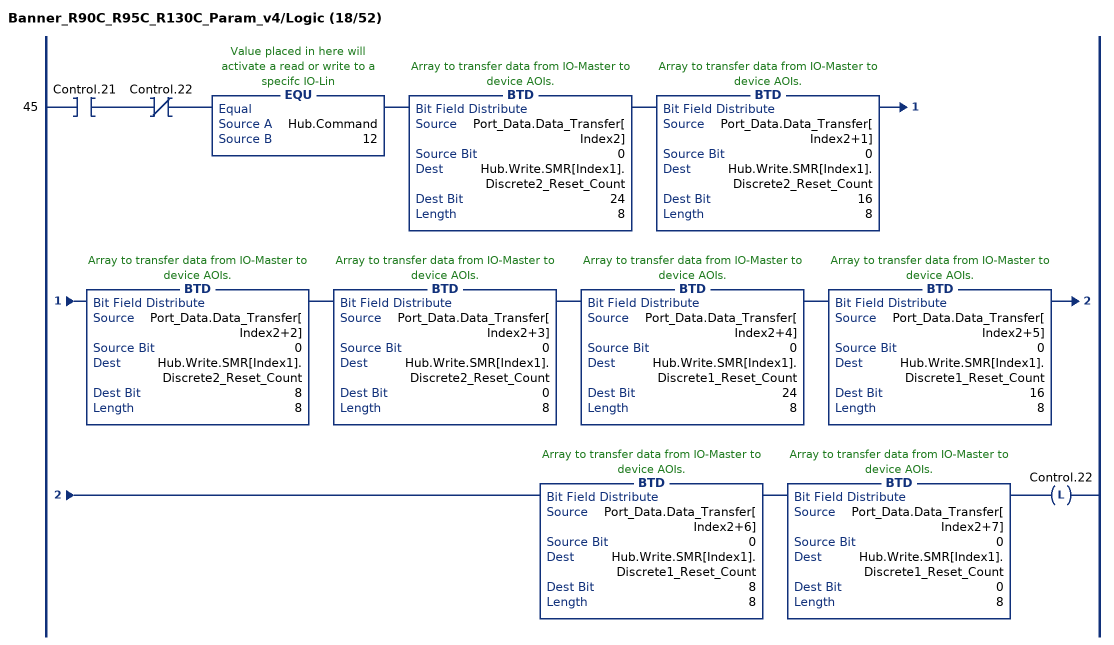
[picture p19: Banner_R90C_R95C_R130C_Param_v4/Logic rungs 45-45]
   45: XIC(Control.21)XIO(Control.22)EQU(Hub.Command,12)BTD(Port_Data.Data_Transfer[Index2],0,Hub.Write.SMR[Index1].Discrete2_Reset_Count,24,8)BTD(Port_Data.Data_Transfer[Index2+1],0,Hub.Write.SMR[Index1].Discrete2_Reset_Count,16,8)BTD(Port_Data.Data_Transfer[Index2+2],0,Hub.Write.SMR[Index1].Discrete2_Reset_Count,8,8)BTD(Port_Data.Data_Transfer[Index2+3],0,Hub.Write.SMR[Index1].Discrete2_Reset_Count,0,8)BTD(Port_Data.Data_Transfer[Index2+4],0,Hub.Write.SMR[Index1].Discrete1_Reset_Count,24,8)BTD(Port_Data.Data_Transfer[Index2+5],0,Hub.Write.SMR[Index1].Discrete1_Reset_Count,16,8)BTD(Port_Data.Data_Transfer[Index2+6],0,Hub.Write.SMR[Index1].Discrete1_Reset_Count,8,8)BTD(Port_Data.Data_Transfer[Index2+7],0,Hub.Write.SMR[Index1].Discrete1_Reset_Count,0,8)OTL(Control.22);
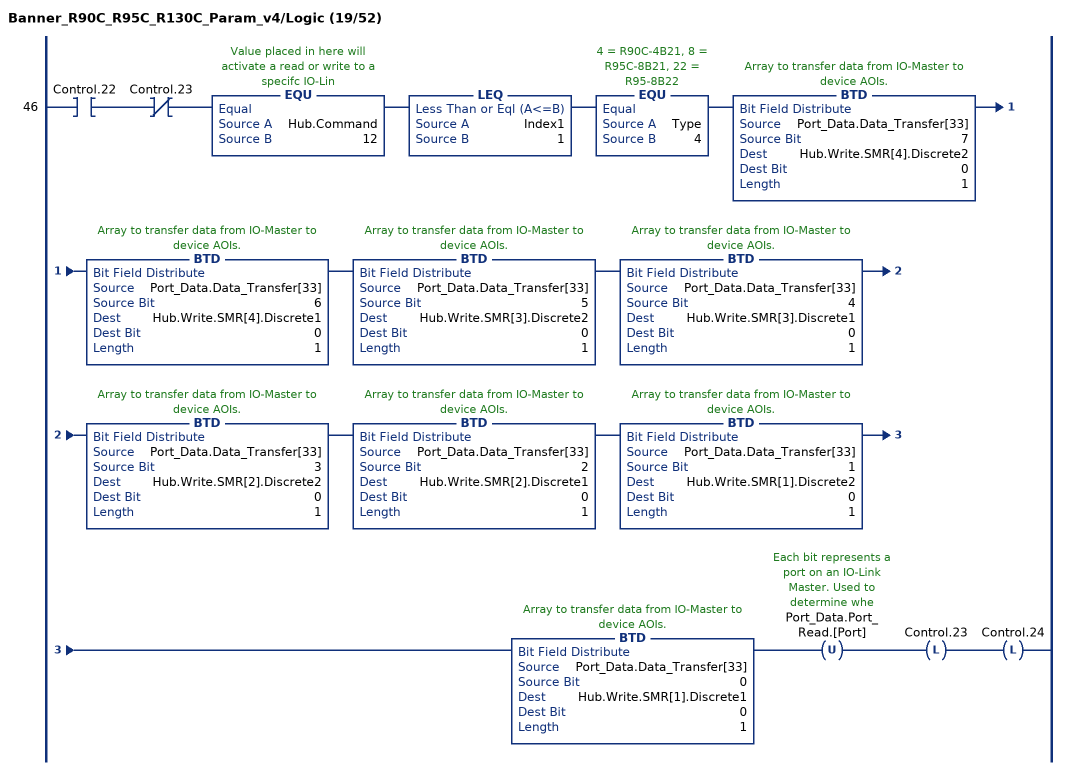
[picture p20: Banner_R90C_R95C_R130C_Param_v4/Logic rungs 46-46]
   46: XIC(Control.22)XIO(Control.23)EQU(Hub.Command,12)LEQ(Index1,1)EQU(Type,4)BTD(Port_Data.Data_Transfer[33],7,Hub.Write.SMR[4].Discrete2,0,1)BTD(Port_Data.Data_Transfer[33],6,Hub.Write.SMR[4].Discrete1,0,1)BTD(Port_Data.Data_Transfer[33],5,Hub.Write.SMR[3].Discrete2,0,1)BTD(Port_Data.Data_Transfer[33],4,Hub.Write.SMR[3].Discrete1,0,1)BTD(Port_Data.Data_Transfer[33],3,Hub.Write.SMR[2].Discrete2,0,1)BTD(Port_Data.Data_Transfer[33],2,Hub.Write.SMR[2].Discrete1,0,1)BTD(Port_Data.Data_Transfer[33],1,Hub.Write.SMR[1].Discrete2,0,1)BTD(Port_Data.Data_Transfer[33],0,Hub.Write.SMR[1].Discrete1,0,1)OTU(Port_Data.Port_Read.[Port])OTL(Control.23)OTL(Control.24);
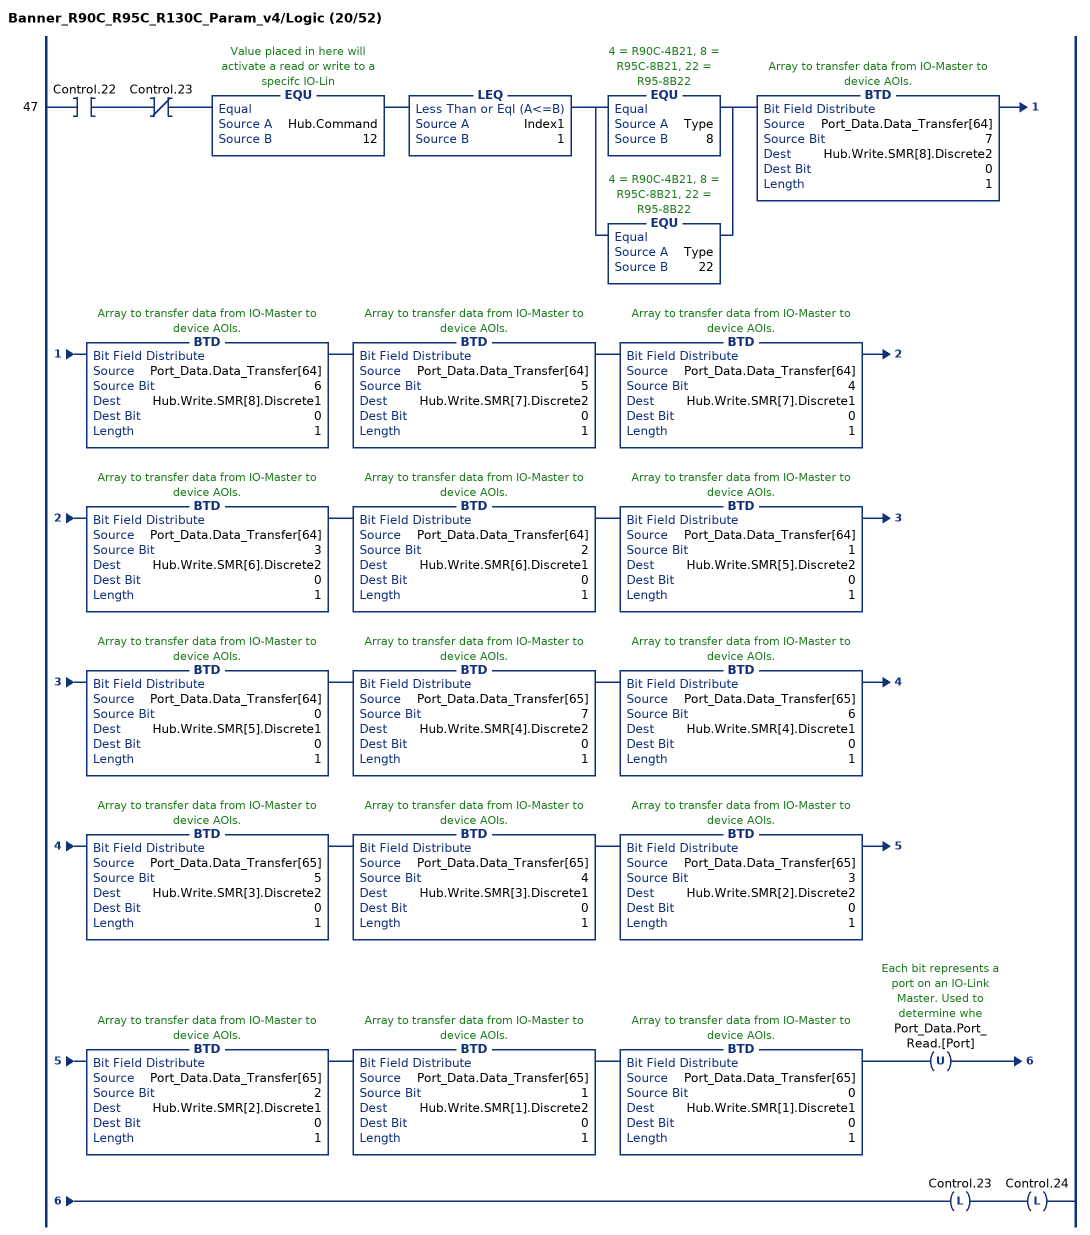
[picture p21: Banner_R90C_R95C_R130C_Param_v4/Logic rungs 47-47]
   47: XIC(Control.22)XIO(Control.23)EQU(Hub.Command,12)LEQ(Index1,1)[EQU(Type,8) ,EQU(Type,22) ]BTD(Port_Data.Data_Transfer[64],7,Hub.Write.SMR[8].Discrete2,0,1)BTD(Port_Data.Data_Transfer[64],6,Hub.Write.SMR[8].Discrete1,0,1)BTD(Port_Data.Data_Transfer[64],5,Hub.Write.SMR[7].Discrete2,0,1)BTD(Port_Data.Data_Transfer[64],4,Hub.Write.SMR[7].Discrete1,0,1)BTD(Port_Data.Data_Transfer[64],3,Hub.Write.SMR[6].Discrete2,0,1)BTD(Port_Data.Data_Transfer[64],2,Hub.Write.SMR[6].Discrete1,0,1)BTD(Port_Data.Data_Transfer[64],1,Hub.Write.SMR[5].Discrete2,0,1)BTD(Port_Data.Data_Transfer[64],0,Hub.Write.SMR[5].Discrete1,0,1)BTD(Port_Data.Data_Transfer[65],7,Hub.Write.SMR[4].Discrete2,0,1)BTD(Port_Data.Data_Transfer[65],6,Hub.Write.SMR[4].Discrete1,0,1)BTD(Port_Data.Data_Transfer[65],5,Hub.Write.SMR[3].Discrete2,0,1)BTD(Port_Data.Data_Transfer[65],4,Hub.Write.SMR[3].Discrete1,0,1)BTD(Port_Data.Data_Transfer[65],3,Hub.Write.SMR[2].Discrete2,0,1)BTD(Port_Data.Data_Transfer[65],2,Hub.Write.SMR[2].Discrete1,0,1)BTD(Port_Data.Data_Transfer[65],1,Hub.Write.SMR[1].Discrete2,0,1)BTD(Port_Data.Data_Transfer[65],0,Hub.Write.SMR[1].Discrete1,0,1)OTU(Port_Data.Port_Read.[Port])OTL(Control.23)OTL(Control.24);
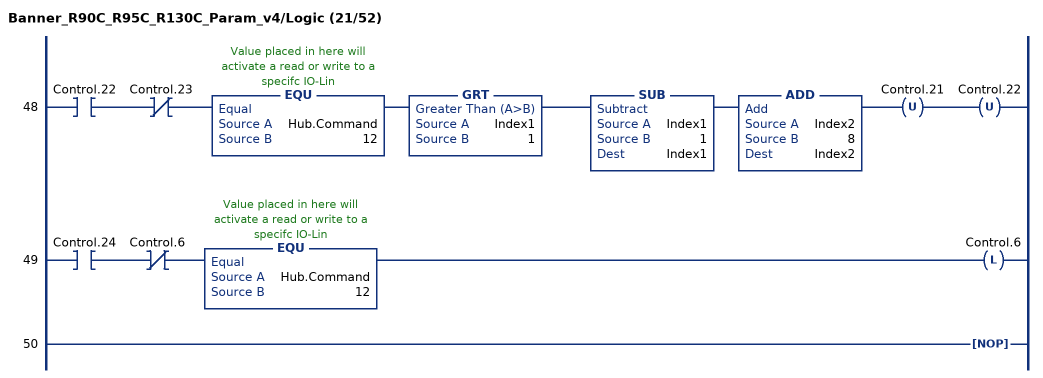
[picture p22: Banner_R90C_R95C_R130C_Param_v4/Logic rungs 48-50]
   48: XIC(Control.22)XIO(Control.23)EQU(Hub.Command,12)GRT(Index1,1)SUB(Index1,1,Index1)ADD(Index2,8,Index2)OTU(Control.21)OTU(Control.22);
   49: XIC(Control.24)XIO(Control.6)EQU(Hub.Command,12)OTL(Control.6);
   50: NOP();
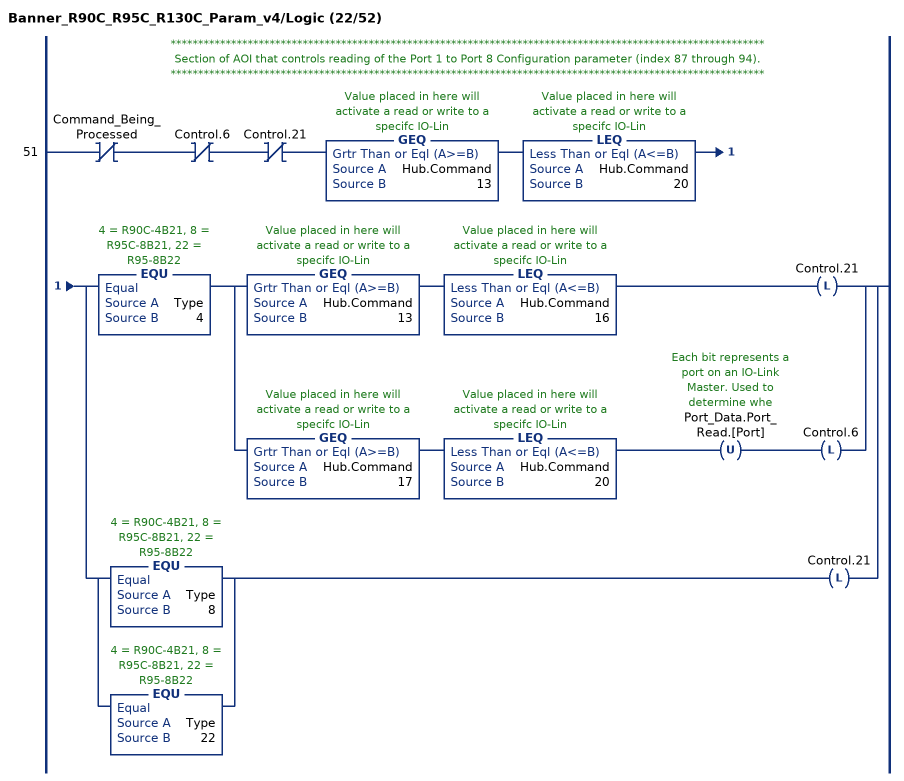
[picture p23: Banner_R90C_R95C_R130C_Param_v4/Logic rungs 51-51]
   // ************************************************************************************************************
   // Section of AOI that controls reading of the Port 1 to Port 8 Configuration parameter (index 87 through 94).
   // ************************************************************************************************************
   51: XIO(Command_Being_Processed)XIO(Control.6)XIO(Control.21)GEQ(Hub.Command,13)LEQ(Hub.Command,20)[EQU(Type,4) [GEQ(Hub.Command,13) LEQ(Hub.Command,16) OTL(Control.21) ,GEQ(Hub.Command,17) LEQ(Hub.Command,20) OTU(Port_Data.Port_Read.[Port]) OTL(Control.6) ] ,[EQU(Type,8) ,EQU(Type,22) ] OTL(Control.21) ];
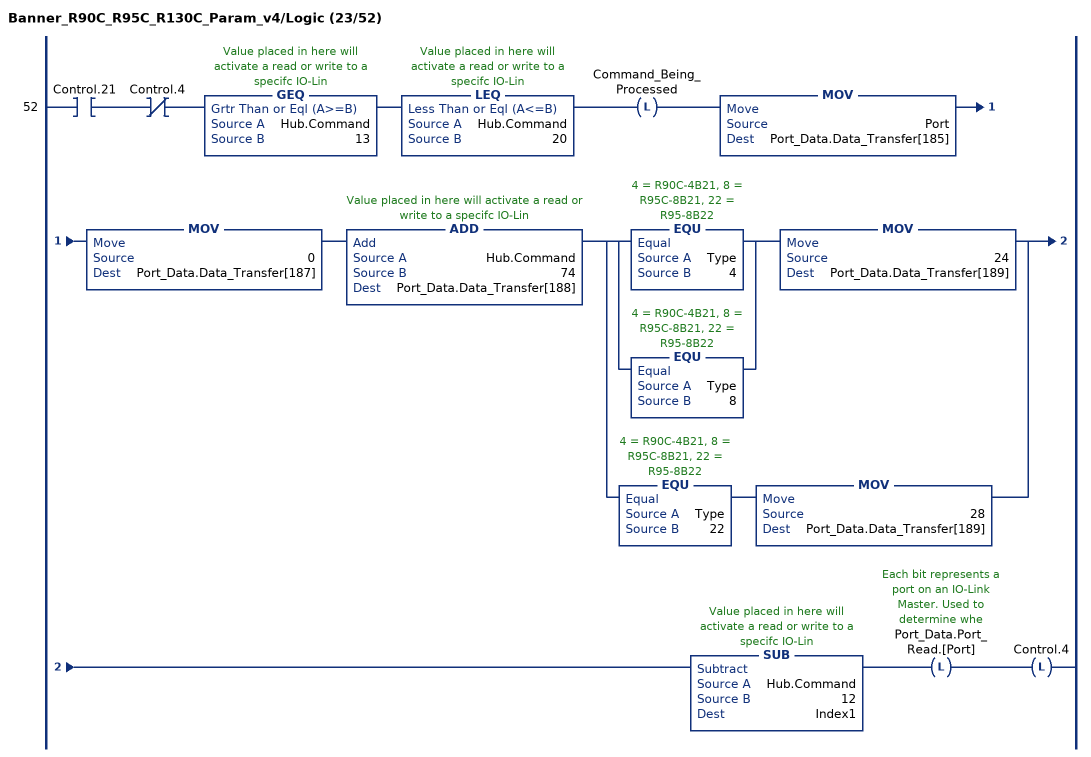
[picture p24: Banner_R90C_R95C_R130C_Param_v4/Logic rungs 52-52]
   52: XIC(Control.21)XIO(Control.4)GEQ(Hub.Command,13)LEQ(Hub.Command,20)OTL(Command_Being_Processed)MOV(Port,Port_Data.Data_Transfer[185])MOV(0,Port_Data.Data_Transfer[187])ADD(Hub.Command,74,Port_Data.Data_Transfer[188])[[EQU(Type,4) ,EQU(Type,8) ] MOV(24,Port_Data.Data_Transfer[189]) ,EQU(Type,22) MOV(28,Port_Data.Data_Transfer[189]) ]SUB(Hub.Command,12,Index1)OTL(Port_Data.Port_Read.[Port])OTL(Control.4);
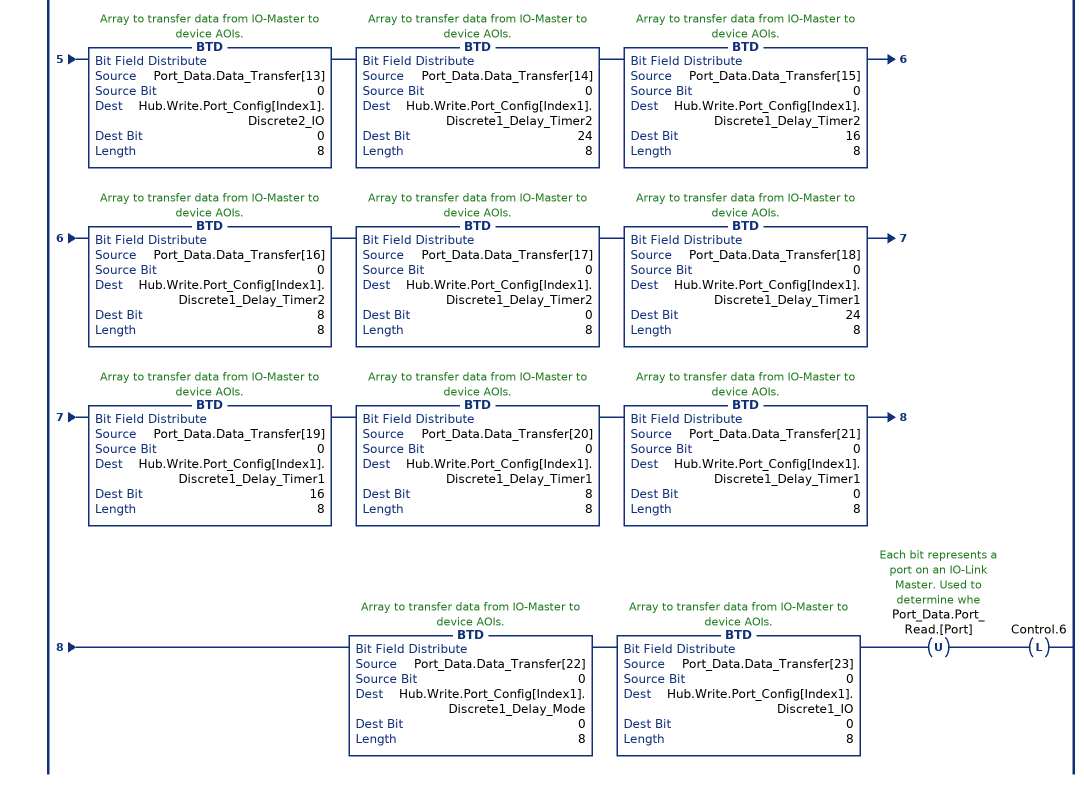
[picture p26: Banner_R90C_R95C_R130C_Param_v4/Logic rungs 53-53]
   53: XIC(Control.5)XIO(Control.6)GEQ(Hub.Command,13)LEQ(Hub.Command,20)[EQU(Type,4) ,EQU(Type,8) ]BTD(Port_Data.Data_Transfer[0],0,Hub.Write.Port_Config[Index1].Mirroring_Inversion,0,8)BTD(Port_Data.Data_Transfer[1],0,Hub.Write.Port_Config[Index1].Mirroring_Channel,0,8)BTD(Port_Data.Data_Transfer[2],0,Hub.Write.Port_Config[Index1].Mirroring_Port,0,8)BTD(Port_Data.Data_Transfer[3],0,Hub.Write.Port_Config[Index1].Mirroring_Enable,0,8)BTD(Port_Data.Data_Transfer[4],0,Hub.Write.Port_Config[Index1].Discrete2_Delay_Timer2,24,8)BTD(Port_Data.Data_Transfer[5],0,Hub.Write.Port_Config[Index1].Discrete2_Delay_Timer2,16,8)BTD(Port_Data.Data_Transfer[6],0,Hub.Write.Port_Config[Index1].Discrete2_Delay_Timer2,8,8)BTD(Port_Data.Data_Transfer[7],0,Hub.Write.Port_Config[Index1].Discrete2_Delay_Timer2,0,8)BTD(Port_Data.Data_Transfer[8],0,Hub.Write.Port_Config[Index1].Discrete2_Delay_Timer1,24,8)BTD(Port_Data.Data_Transfer[9],0,Hub.Write.Port_Config[Index1].Discrete2_Delay_Timer1,16,8)BTD(Port_Data.Data_Transfer[10],0,Hub.Write.Port_Config[Index1].Discrete2_Delay_Timer1,8,8)BTD(Port_Data.Data_Transfer[11],0,Hub.Write.Port_Config[Index1].Discrete2_Delay_Timer1,0,8)BTD(Port_Data.Data_Transfer[12],0,Hub.Write.Port_Config[Index1].Discrete2_Delay_Mode,0,8)BTD(Port_Data.Data_Transfer[13],0,Hub.Write.Port_Config[Index1].Discrete2_IO,0,8)BTD(Port_Data.Data_Transfer[14],0,Hub.Write.Port_Config[Index1].Discrete1_Delay_Timer2,24,8)BTD(Port_Data.Data_Transfer[15],0,Hub.Write.Port_Config[Index1].Discrete1_Delay_Timer2,16,8)BTD(Port_Data.Data_Transfer[16],0,Hub.Write.Port_Config[Index1].Discrete1_Delay_Timer2,8,8)BTD(Port_Data.Data_Transfer[17],0,Hub.Write.Port_Config[Index1].Discrete1_Delay_Timer2,0,8)BTD(Port_Data.Data_Transfer[18],0,Hub.Write.Port_Config[Index1].Discrete1_Delay_Timer1,24,8)BTD(Port_Data.Data_Transfer[19],0,Hub.Write.Port_Config[Index1].Discrete1_Delay_Timer1,16,8)BTD(Port_Data.Data_Transfer[20],0,Hub.Write.Port_Config[Index1].Discrete1_Delay_Timer1,8,8)BTD(Port_Data.Data_Transfer[21],0,Hub.Write.Port_Config[Index1].Discrete1_Delay_Timer1,0,8)BTD(Port_Data.Data_Transfer[22],0,Hub.Write.Port_Config[Index1].Discrete1_Delay_Mode,0,8)BTD(Port_Data.Data_Transfer[23],0,Hub.Write.Port_Config[Index1].Discrete1_IO,0,8)OTU(Port_Data.Port_Read.[Port])OTL(Control.6);
